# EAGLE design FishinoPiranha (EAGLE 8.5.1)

## Sheet 1 of 6: SUPPLY
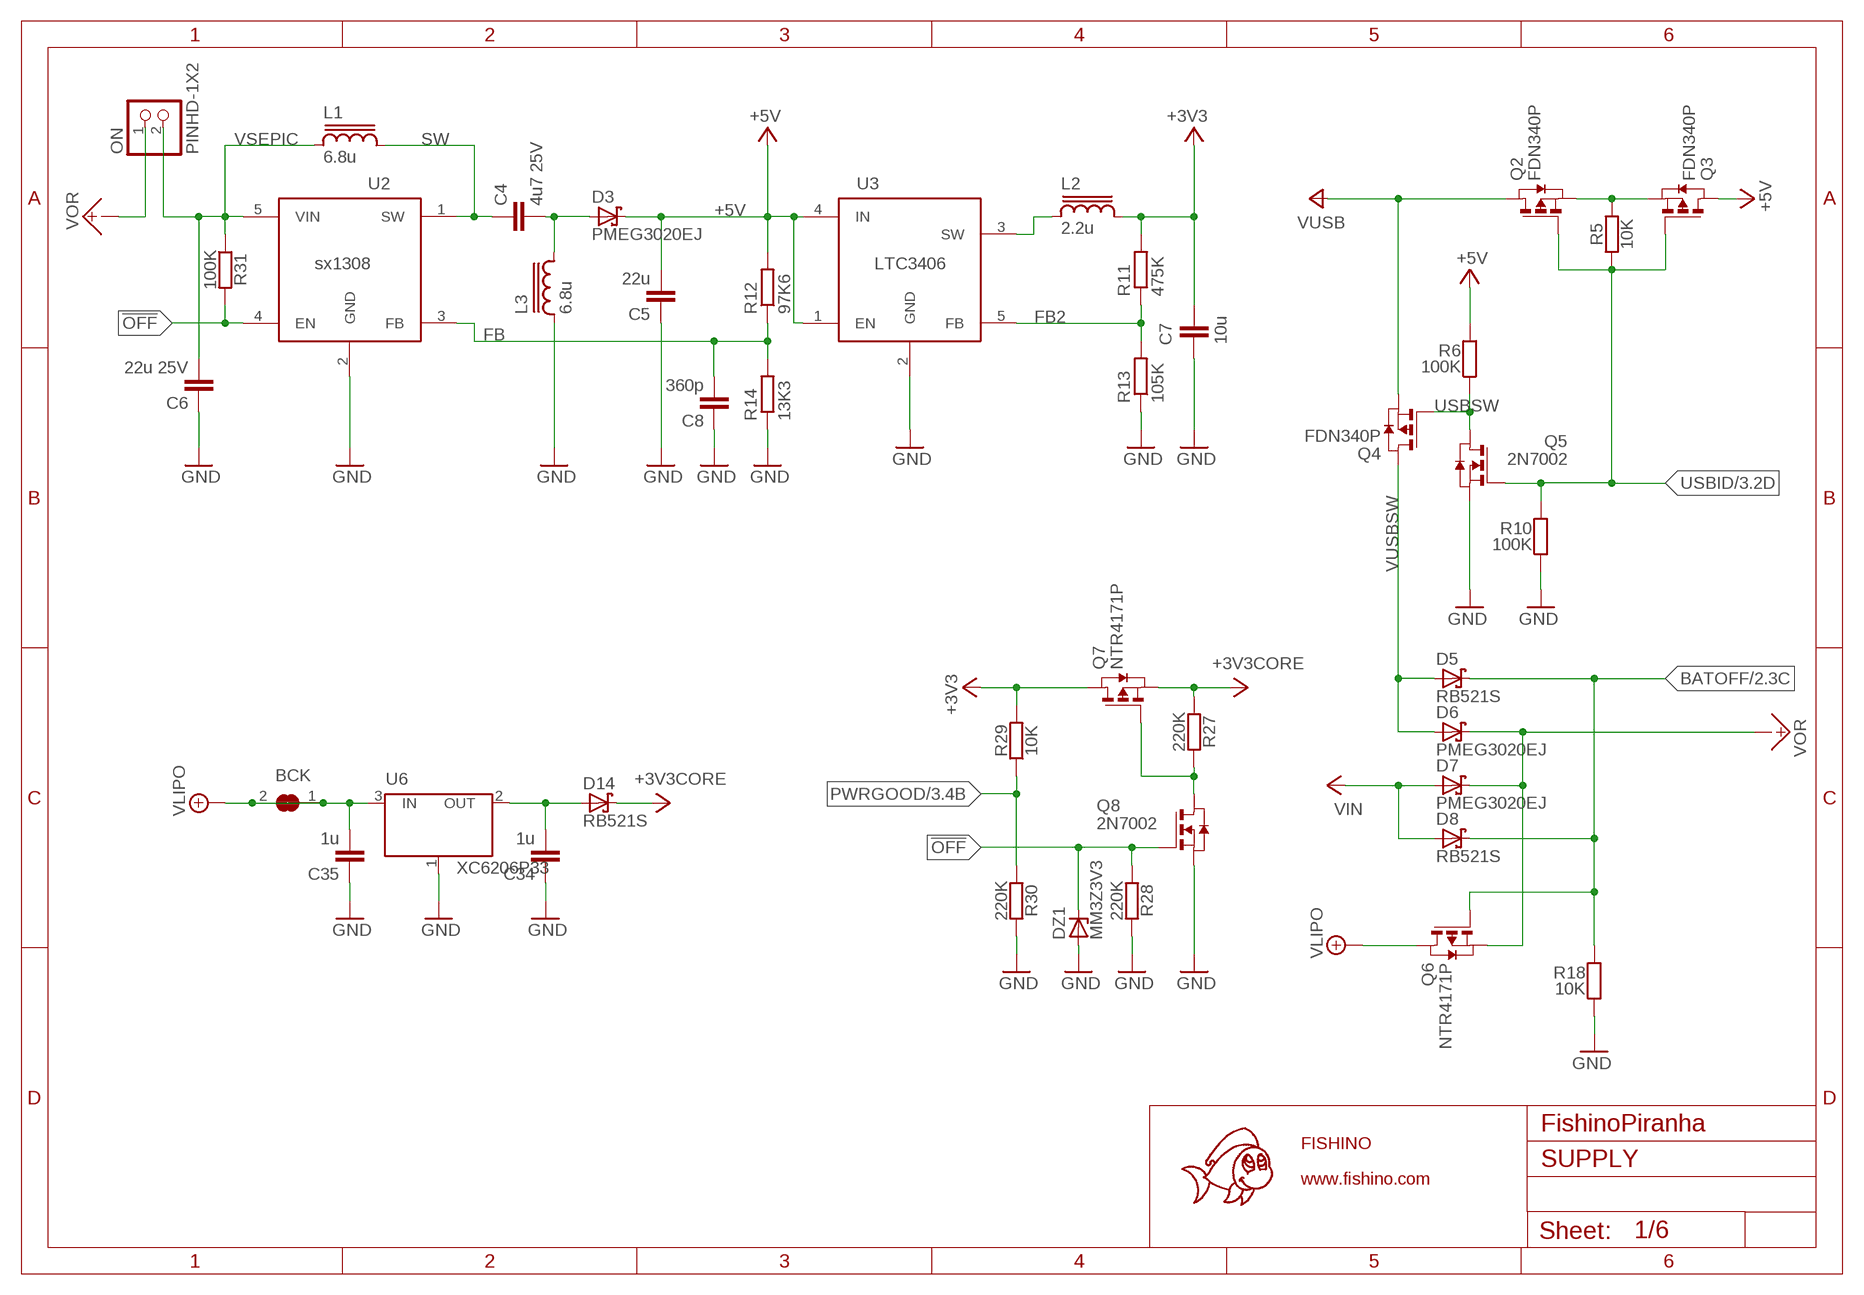
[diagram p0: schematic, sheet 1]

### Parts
BCK  SJ  [SJ]
C4  4u7 25V  C0603-ROUND  [C0603-ROUND]
C5  22u  C0603-ROUND  [C0603-ROUND]
C6  22u 25V  C0603-ROUND  [C0603-ROUND]
C7  10u  C0603-ROUND  [C0603-ROUND]
C8  360p  C0603-ROUND  [C0603-ROUND]
C34  1u  C0603-ROUND  [C0603-ROUND]
C35  1u  C0603-ROUND  [C0603-ROUND]
D3  PMEG3020EJ  [SOD-323]
D5  RB521S  [SOD523]
D6  PMEG3020EJ  [SOD-323]
D7  PMEG3020EJ  [SOD-323]
D8  RB521S  [SOD523]
D14  RB521S  [SOD523]
DZ1  MM3Z3V3  [SOD-323]
L1  6.8u  LSWPA4030S  [SWPA4030S]
L2  2.2u  LCD32  [CD32]
L3  6.8u  LSWPA4030S  [SWPA4030S]
ON  PINHD-1X2  [1X02M]
Q2  FDN340P  PMOSSOT23  [SOT23]
Q3  FDN340P  PMOSSOT23  [SOT23]
Q4  FDN340P  PMOSSOT23  [SOT23]
Q5  2N7002  [SOT23]
Q6  NTR4171P  [SOT23]
Q7  NTR4171P  [SOT23]
Q8  2N7002  [SOT23]
R5  10K  R0603-ROUND  [R0603-ROUND]
R6  100K  R0603-ROUND  [R0603-ROUND]
R10  100K  R0603-ROUND  [R0603-ROUND]
R11  475K  R0603-ROUND  [R0603-ROUND]
R12  97K6  R0603-ROUND  [R0603-ROUND]
R13  105K  R0603-ROUND  [R0603-ROUND]
R14  13K3  R0603-ROUND  [R0603-ROUND]
R18  10K  R0603-ROUND  [R0603-ROUND]
R27  220K  R0603-ROUND  [R0603-ROUND]
R28  220K  R0603-ROUND  [R0603-ROUND]
R29  10K  R0603-ROUND  [R0603-ROUND]
R30  220K  R0603-ROUND  [R0603-ROUND]
R31  100K  R0603-ROUND  [R0603-ROUND]
U2  SX1308  [SOT23-6L]
U3  LC3406  [SOT23-5]
U6  XC6206P33  [SOT23-3]

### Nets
!OFF: DZ1.C Q8.1(G) R28.1 R31.2 U2.4(EN) ; also sheet 3
+3V3: C7.2 L2.2 Q7.3(D) R11.2 R29.2 ; also sheet 3,4,5,6
+3V3CORE: D14.C Q7.2(S) R27.1 ; also sheet 3,5,6
+5V: C5.2 D3.C Q3.3(D) R6.2 R12.2 U3.1(EN) U3.4(IN) ; also sheet 2,6
BATOFF: D5.C D8.C Q6.1(G) R18.2 ; also sheet 2
FB: C8.2 R12.1 R14.2 U2.3(FB)
FB2: R11.1 R13.2 U3.5(FB)
GND [gnd]: C5.1 C6.1 C7.1 C8.1 C34.1 C35.1 DZ1.A L3.P$1 Q5.2(S) Q8.2(S) R10.1 R13.1 R14.1 R18.1 R28.2 R30.2 U2.2(GND) U3.2(GND) U6.1(GND/ADJ) ; also sheet 2,3,4,5,6
N17690335: Q2.2(S) Q3.2(S) R5.2
N$1: C34.2 D14.A U6.2(OUT)
N$24: C4.2 D3.A L3.P$2
N$34: Q7.1(G) Q8.3(D) R27.2
PWRGOOD: R29.1 R30.1 ; also sheet 3
SW: C4.1 L1.P$2 U2.1(SW)
SW2: L2.1 U3.3(SW)
USBID: Q2.1(G) Q3.1(G) Q5.1(G) R5.1 R10.2 ; also sheet 3,6
USBSW: Q4.1(G) Q5.3(D) R6.1
VIN: D7.A D8.A ; also sheet 6
VLIPO: BCK.1 BCK.2 C35.2 Q6.3(D) U6.3(IN) ; also sheet 2
VOR [power]: D6.C D7.C ON.1 Q6.2(S)
VSEPIC [power]: C6.2 L1.P$1 ON.2 R31.1 U2.5(VIN)
VUSB: Q2.3(D) Q4.2(S) ; also sheet 3,6
VUSBSW: D5.A D6.A Q4.3(D)

## Sheet 2 of 6: BATTERY CHARGER
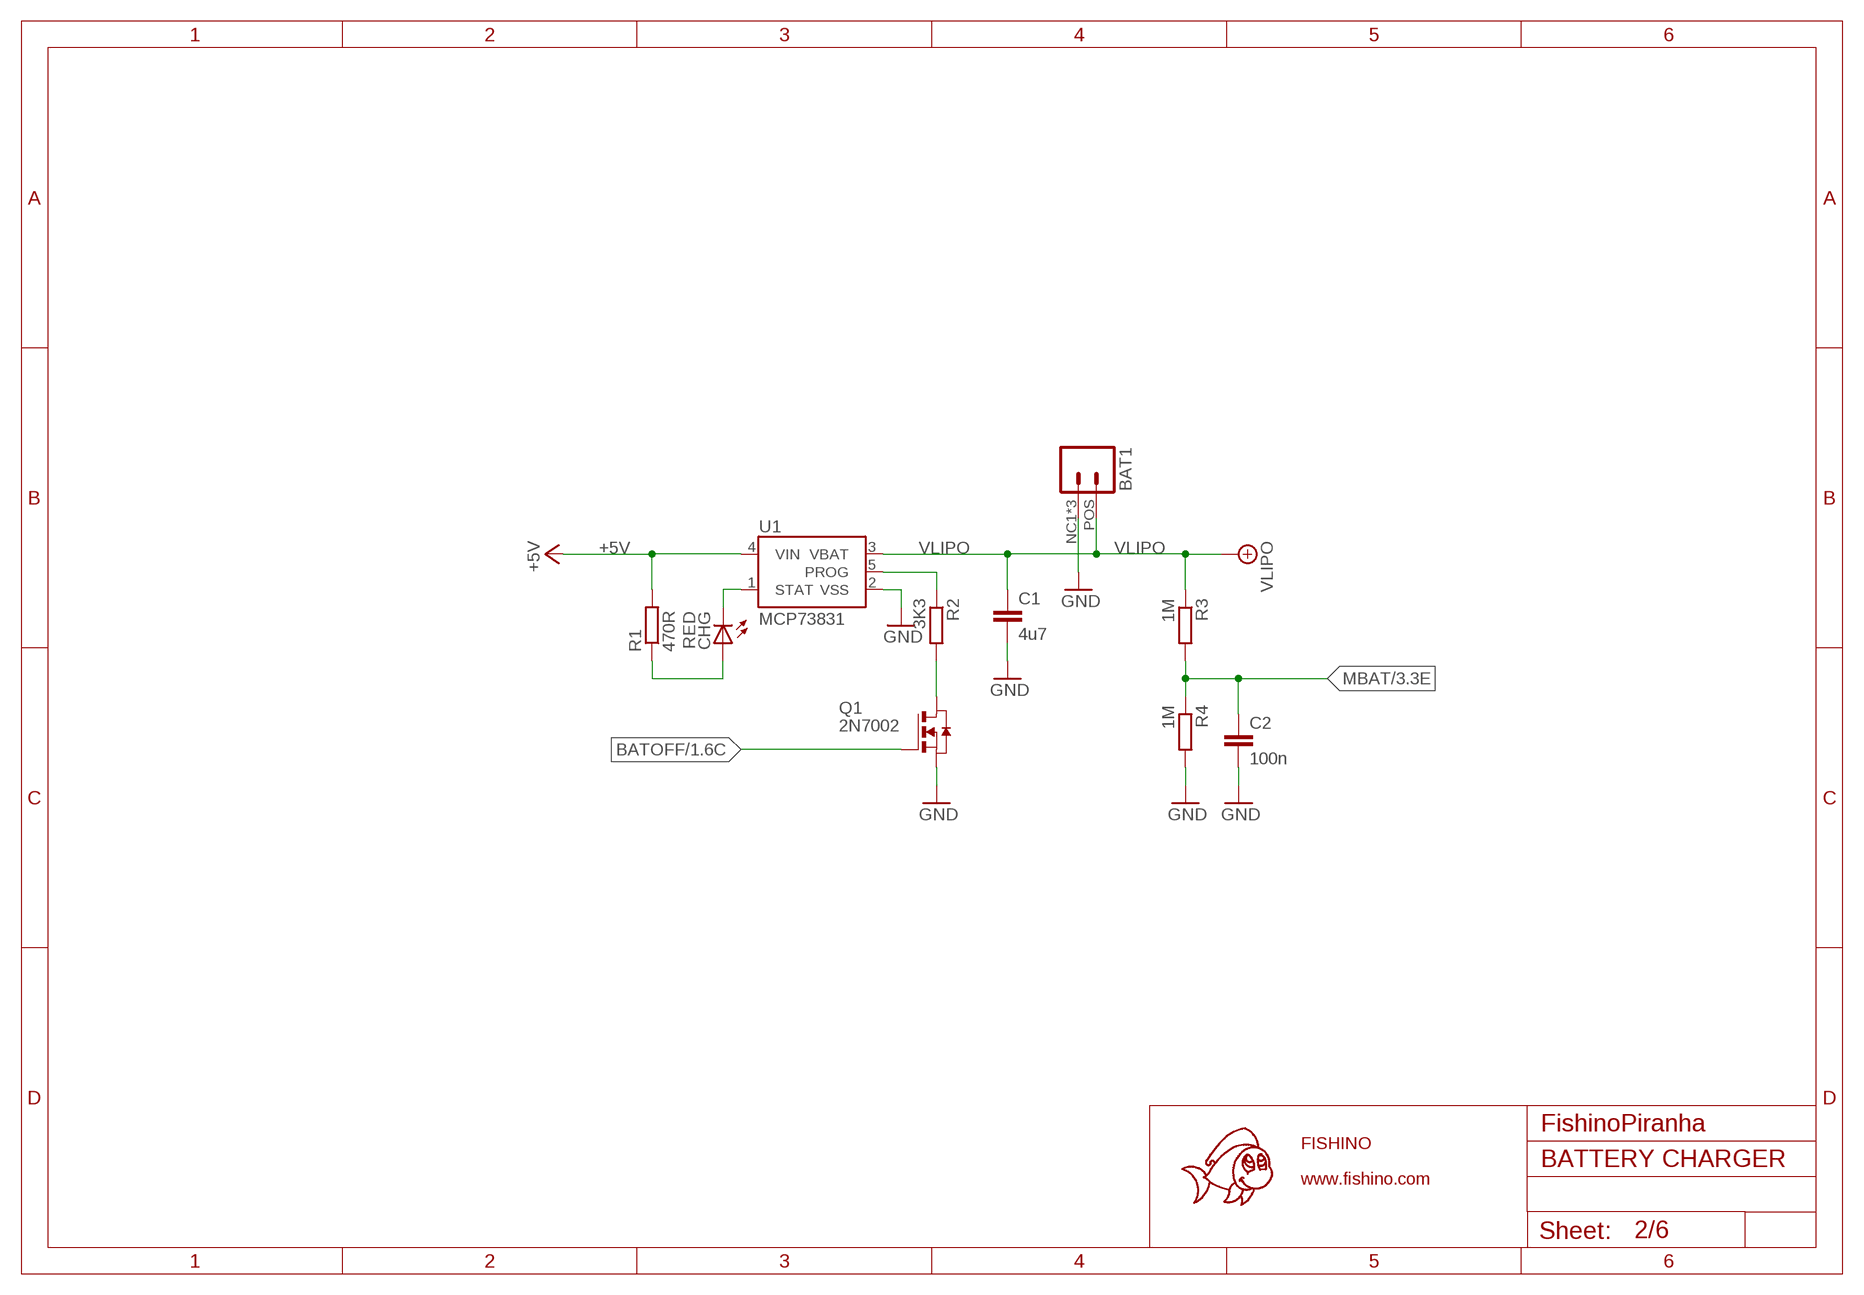
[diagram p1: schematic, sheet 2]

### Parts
BAT1  MO2-JST-2-2MM-SMT-STANDARD  [JST-2-SMD-STANDARD]
C1  4u7  C0603-ROUND  [C0603-ROUND]
C2  100n  C0603-ROUND  [C0603-ROUND]
CHG  RED  LED0603  [CHIPLED_0603]
Q1  2N7002  [SOT23]
R1  470R  R0603-ROUND  [R0603-ROUND]
R2  3K3  R0603-ROUND  [R0603-ROUND]
R3  1M  R0603-ROUND  [R0603-ROUND]
R4  1M  R0603-ROUND  [R0603-ROUND]
U1  MCP73831  [SOT23-5]

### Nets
+5V: R1.2 U1.4(VIN) ; also sheet 1,6
BATOFF: Q1.1(G) ; also sheet 1
GND [gnd]: BAT1.NC1(NEG) BAT1.NC2(NEG) BAT1.NEG C1.2 C2.2 Q1.2(S) R4.2 U1.2(VSS) ; also sheet 1,3,4,5,6
MBAT: C2.1 R3.2 R4.1 ; also sheet 3
N$7: Q1.3(D) R2.2
N$20: CHG.A R1.1
PROG: R2.1 U1.5(PROG)
STAT2: CHG.C U1.1(STAT)
VLIPO: BAT1.POS C1.1 R3.1 U1.3(VBAT) ; also sheet 1

## Sheet 3 of 6: CONTROLLER
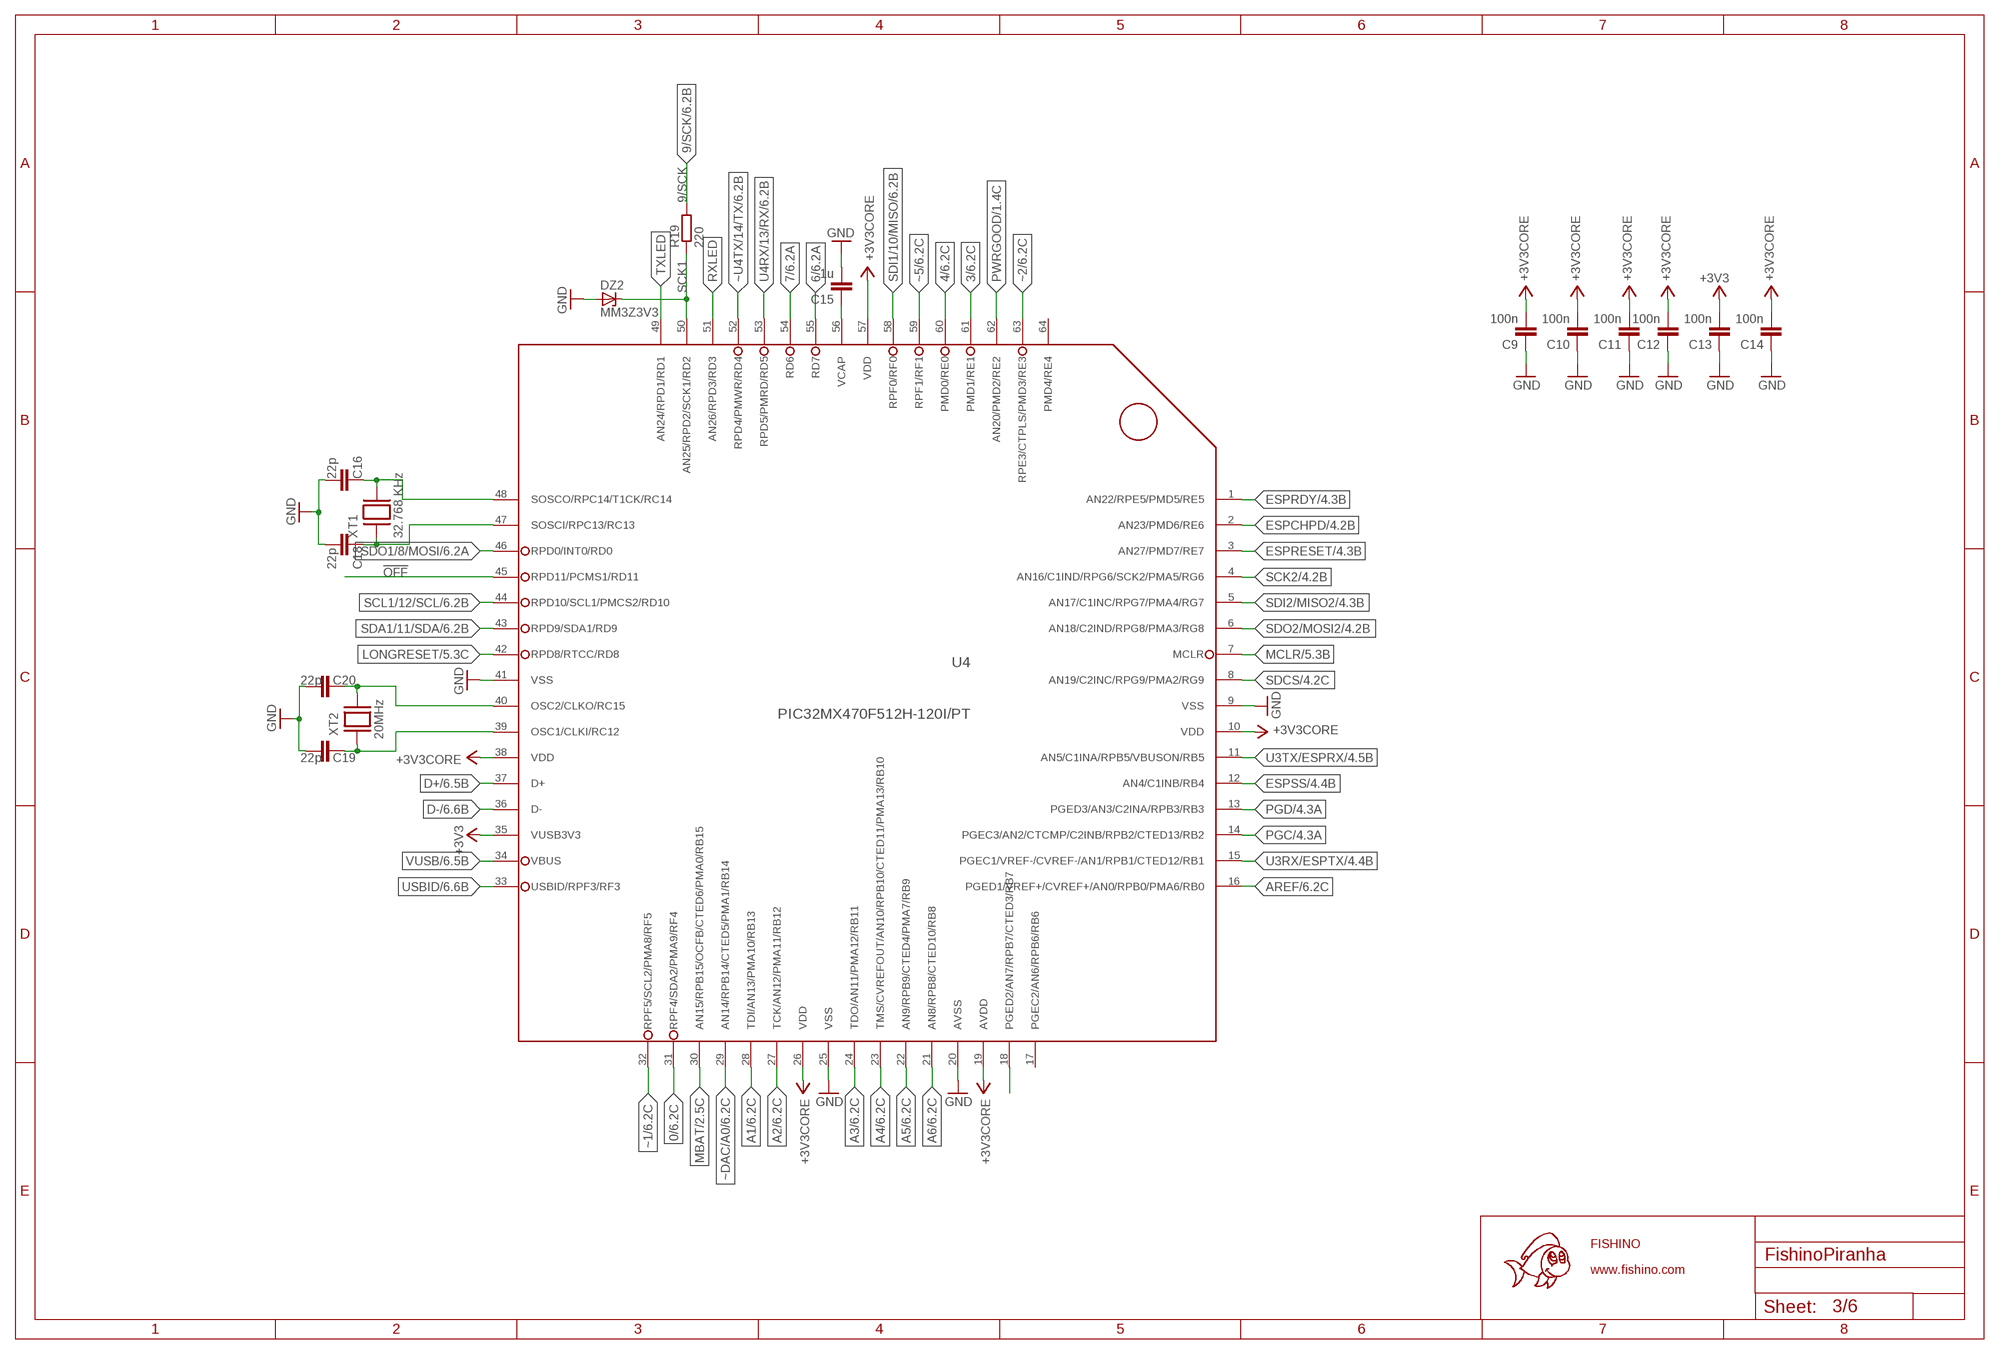
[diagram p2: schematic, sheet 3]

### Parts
C9  100n  C0603-ROUND  [C0603-ROUND]
C10  100n  C0603-ROUND  [C0603-ROUND]
C11  100n  C0603-ROUND  [C0603-ROUND]
C12  100n  C0603-ROUND  [C0603-ROUND]
C13  100n  C0603-ROUND  [C0603-ROUND]
C14  100n  C0603-ROUND  [C0603-ROUND]
C15  1u  C0603-ROUND  [C0603-ROUND]
C16  22p  C0603-ROUND  [C0603-ROUND]
C18  22p  C0603-ROUND  [C0603-ROUND]
C19  22p  C0603-ROUND  [C0603-ROUND]
C20  22p  C0603-ROUND  [C0603-ROUND]
DZ2  MM3Z3V3  [SOD-323]
R19  220  R0603-ROUND  [R0603-ROUND]
U4  PIC32MX470F512H-120I/PT  [TQFP64-10X10]
XT1  32.768 KHz  XTAL/SFC145  [FC145]
XT2  20MHz  XTAL/SIQG2520  [IQG2520]

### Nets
0: U4.31(RPF4/SDA2/PMA9/RF4) ; also sheet 6
3: U4.61(PMD1/RE1) ; also sheet 6
4: U4.60(PMD0/RE0) ; also sheet 6
6: U4.55(RD7) ; also sheet 6
7: U4.54(RD6) ; also sheet 6
9/SCK: R19.2 ; also sheet 6
!OFF: U4.45(RPD11/PCMS1/RD11) ; also sheet 1
+3V3: C13.2 U4.35(VUSB3V3) ; also sheet 1,4,5,6
+3V3CORE: C9.2 C10.2 C11.2 C12.2 C14.2 U4.10(VDD) U4.19(AVDD) U4.26(VDD) U4.38(VDD) U4.57(VDD) ; also sheet 1,5,6
A1: U4.28(TDI/AN13/PMA10/RB13) ; also sheet 6
A2: U4.27(TCK/AN12/PMA11/RB12) ; also sheet 6
A3: U4.24(TDO/AN11/PMA12/RB11) ; also sheet 6
A4: U4.23(TMS/CVREFOUT/AN10/RPB10/CTED11/PMA13/RB10) ; also sheet 6
A5: U4.22(AN9/RPB9/CTED4/PMA7/RB9) ; also sheet 6
A6: U4.21(AN8/RPB8/CTED10/RB8) ; also sheet 6
AREF: U4.16(PGED1/VREF+/CVREF+/AN0/RPB0/PMA6/RB0) ; also sheet 6
D+: U4.37(D+) ; also sheet 6
D-: U4.36(D-) ; also sheet 6
ESPBMODE: U4.18(PGED2/AN7/RPB7/CTED3/RB7) ; also sheet 4
ESPCHPD: U4.2(AN23/PMD6/RE6) ; also sheet 4
ESPRDY: U4.1(AN22/RPE5/PMD5/RE5) ; also sheet 4
ESPRESET: U4.3(AN27/PMD7/RE7) ; also sheet 4
ESPSS: U4.12(AN4/C1INB/RB4) ; also sheet 4
GND [gnd]: C9.1 C10.1 C11.1 C12.1 C13.1 C14.1 C15.2 C16.2 C18.2 C19.2 C20.2 DZ2.A U4.9(VSS) U4.20(AVSS) U4.25(VSS) U4.41(VSS) ; also sheet 1,2,4,5,6
LONGRESET: U4.42(RPD8/RTCC/RD8) ; also sheet 5
MBAT: U4.30(AN15/RPB15/OCFB/CTED6/PMA0/RB15) ; also sheet 2
MCLR: U4.7(MCLR) ; also sheet 5,6
N$2: C15.1 U4.56(VCAP)
N$5: C18.1 U4.47(SOSCI/RPC13/RC13) XT1.P$1
N$6: C16.1 U4.48(SOSCO/RPC14/T1CK/RC14) XT1.P$2
OSC1: C19.1 U4.39(OSC1/CLKI/RC12) XT2.P$3
OSC2: C20.1 U4.40(OSC2/CLKO/RC15) XT2.P$1
PGC: U4.14(PGEC3/AN2/CTCMP/C2INB/RPB2/CTED13/RB2) ; also sheet 4,6
PGD: U4.13(PGED3/AN3/C2INA/RPB3/RB3) ; also sheet 4,6
PWRGOOD: U4.62(AN20/PMD2/RE2) ; also sheet 1
RXLED: U4.51(AN26/RPD3/RD3) ; also sheet 5
SCK1: DZ2.C R19.1 U4.50(AN25/RPD2/SCK1/RD2)
SCK2: U4.4(AN16/C1IND/RPG6/SCK2/PMA5/RG6) ; also sheet 4
SCL1/12/SCL: U4.44(RPD10/SCL1/PMCS2/RD10) ; also sheet 6
SDA1/11/SDA: U4.43(RPD9/SDA1/RD9) ; also sheet 6
SDCS: U4.8(AN19/C2INC/RPG9/PMA2/RG9) ; also sheet 4
SDI1/10/MISO: U4.58(RPF0/RF0) ; also sheet 6
SDI2/MISO2: U4.5(AN17/C1INC/RPG7/PMA4/RG7) ; also sheet 4
SDO1/8/MOSI: U4.46(RPD0/INT0/RD0) ; also sheet 6
SDO2/MOSI2: U4.6(AN18/C2IND/RPG8/PMA3/RG8) ; also sheet 4
TXLED: U4.49(AN24/RPD1/RD1) ; also sheet 5
U3RX/ESPTX: U4.15(PGEC1/VREF-/CVREF-/AN1/RPB1/CTED12/RB1) ; also sheet 4
U3TX/ESPRX: U4.11(AN5/C1INA/RPB5/VBUSON/RB5) ; also sheet 4
U4RX/13/RX: U4.53(RPD5/PMRD/RD5) ; also sheet 6
USBID: U4.33(USBID/RPF3/RF3) ; also sheet 1,6
VUSB: U4.34(VBUS) ; also sheet 1,6
~1: U4.32(RPF5/SCL2/PMA8/RF5) ; also sheet 6
~2: U4.63(RPE3/CTPLS/PMD3/RE3) ; also sheet 6
~5: U4.59(RPF1/RF1) ; also sheet 6
~DAC/A0: U4.29(AN14/RPB14/CTED5/PMA1/RB14) ; also sheet 6
~U4TX/14/TX: U4.52(RPD4/PMWR/RD4) ; also sheet 6
Unconnected: U4.17(PGEC2/AN6/RPB6/RB6) U4.64(PMD4/RE4)

## Sheet 4 of 6: WIFI AND SD
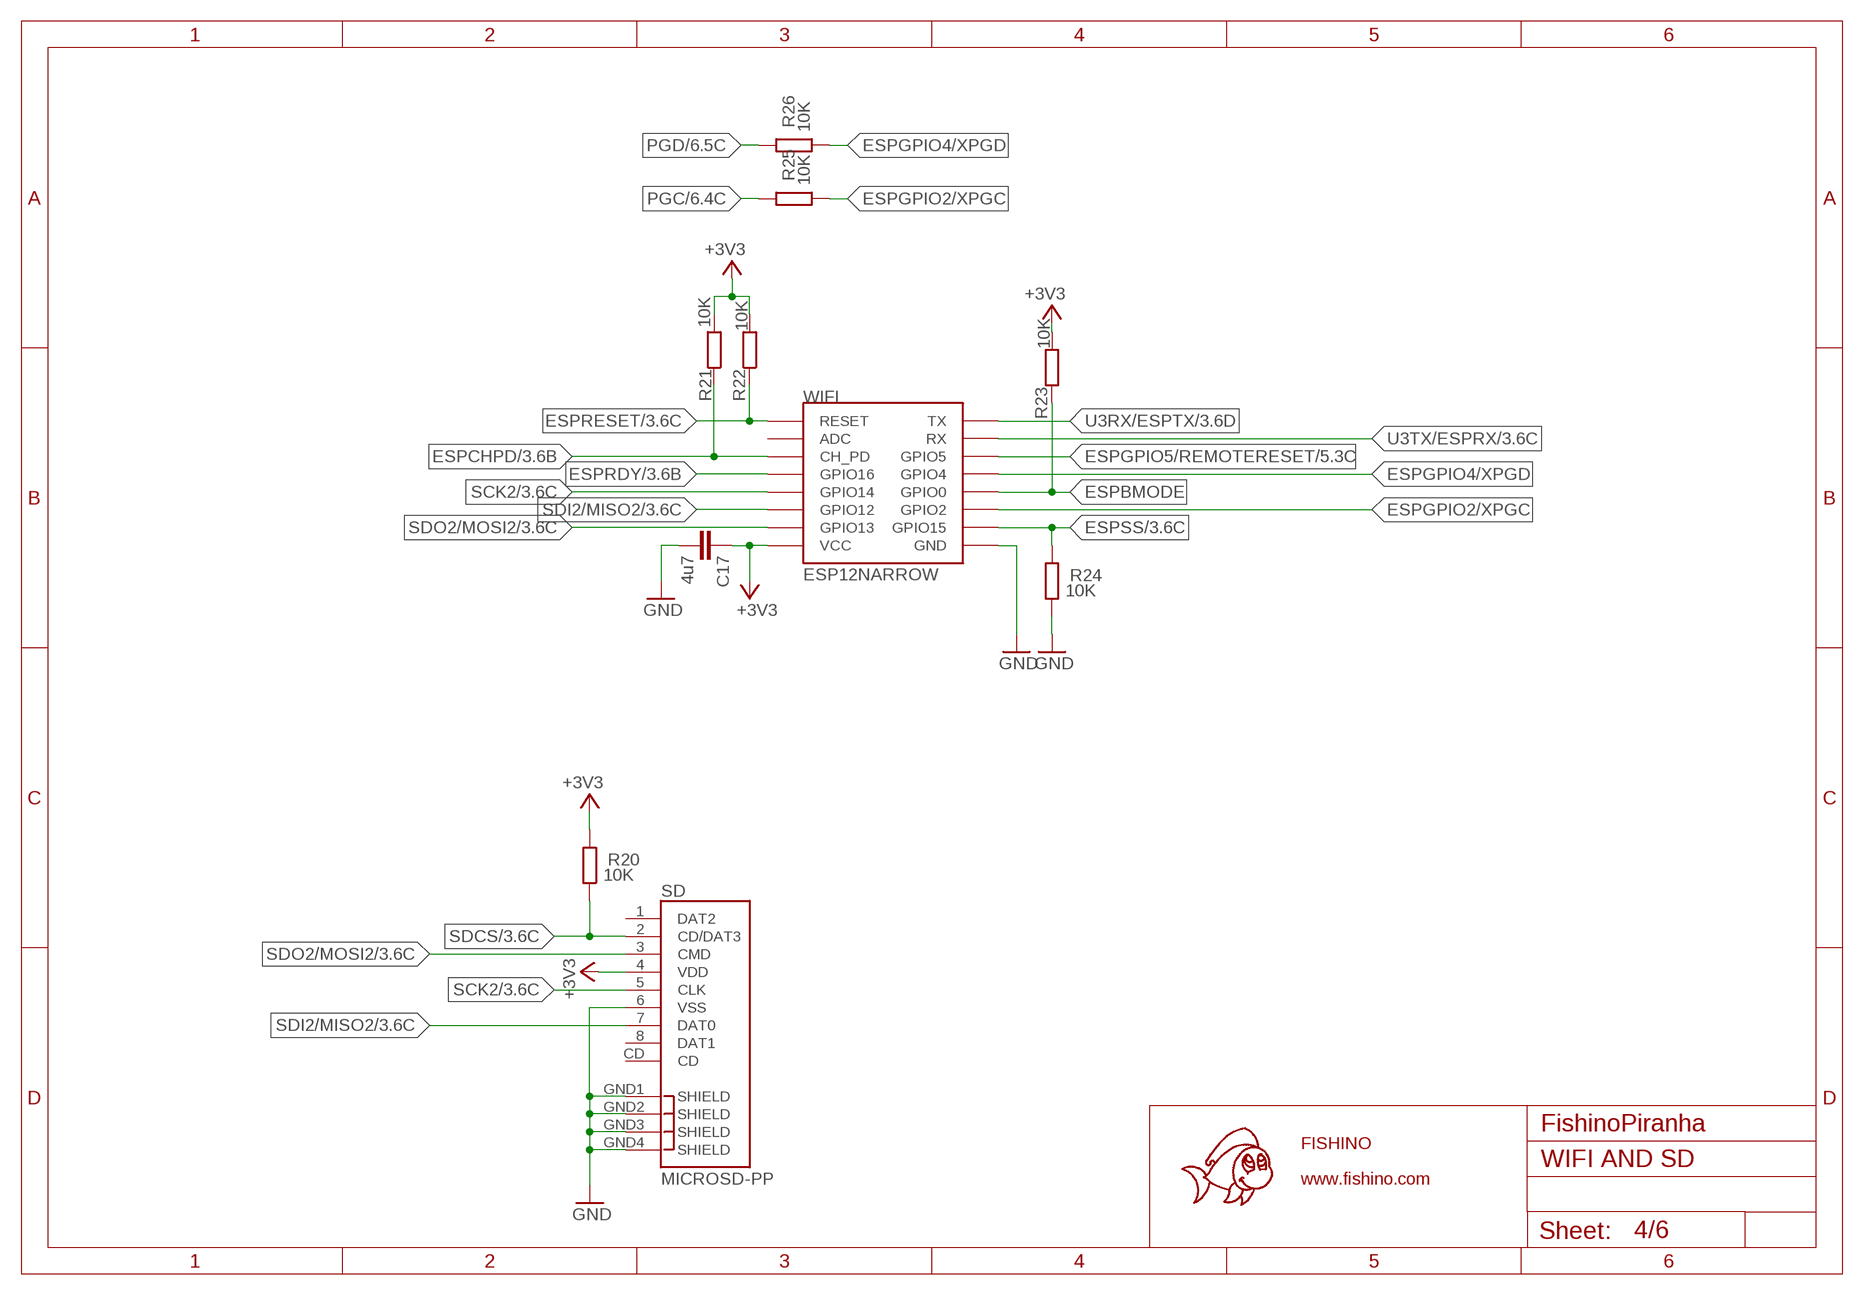
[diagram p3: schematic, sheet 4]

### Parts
C17  4u7  C0603-ROUND  [C0603-ROUND]
R20  10K  R0603-ROUND  [R0603-ROUND]
R21  10K  R0603-ROUND  [R0603-ROUND]
R22  10K  R0603-ROUND  [R0603-ROUND]
R23  10K  R0603-ROUND  [R0603-ROUND]
R24  10K  R0603-ROUND  [R0603-ROUND]
R25  10K  R0603-ROUND  [R0603-ROUND]
R26  10K  R0603-ROUND  [R0603-ROUND]
SD  MICROSD-PP  [MICROSD-PUSHPULL]
WIFI  ESP12NARROW  [ESP12SMD-NARROW]

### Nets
+3V3: C17.1 R20.2 R21.2 R22.2 R23.2 SD.4(VDD) WIFI.VCC ; also sheet 1,3,5,6
ESPBMODE: R23.1 WIFI.GPIO0 ; also sheet 3
ESPCHPD: R21.1 WIFI.CH_PD ; also sheet 3
ESPGPIO2/XPGC: R25.1 WIFI.GPIO2
ESPGPIO4/XPGD: R26.1 WIFI.GPIO4
ESPGPIO5/REMOTERESET: WIFI.GPIO5 ; also sheet 5
ESPRDY: WIFI.GPIO16 ; also sheet 3
ESPRESET: R22.1 WIFI.RESET ; also sheet 3
ESPSS: R24.2 WIFI.GPIO15 ; also sheet 3
GND [gnd]: C17.2 R24.1 SD.6(VSS) SD.GND1(SHIELD) SD.GND2(SHIELD) SD.GND3(SHIELD) SD.GND4(SHIELD) WIFI.GND ; also sheet 1,2,3,5,6
PGC: R25.2 ; also sheet 3,6
PGD: R26.2 ; also sheet 3,6
SCK2: SD.5(CLK) WIFI.GPIO14 ; also sheet 3
SDCS: R20.1 SD.2(CD/DAT3) ; also sheet 3
SDI2/MISO2: SD.7(DAT0) WIFI.GPIO12 ; also sheet 3
SDO2/MOSI2: SD.3(CMD) WIFI.GPIO13 ; also sheet 3
U3RX/ESPTX: WIFI.TX ; also sheet 3
U3TX/ESPRX: WIFI.RX ; also sheet 3
Unconnected: SD.1(DAT2) SD.8(DAT1) SD.CD WIFI.ADC

## Sheet 5 of 6: RESET AND LEDS
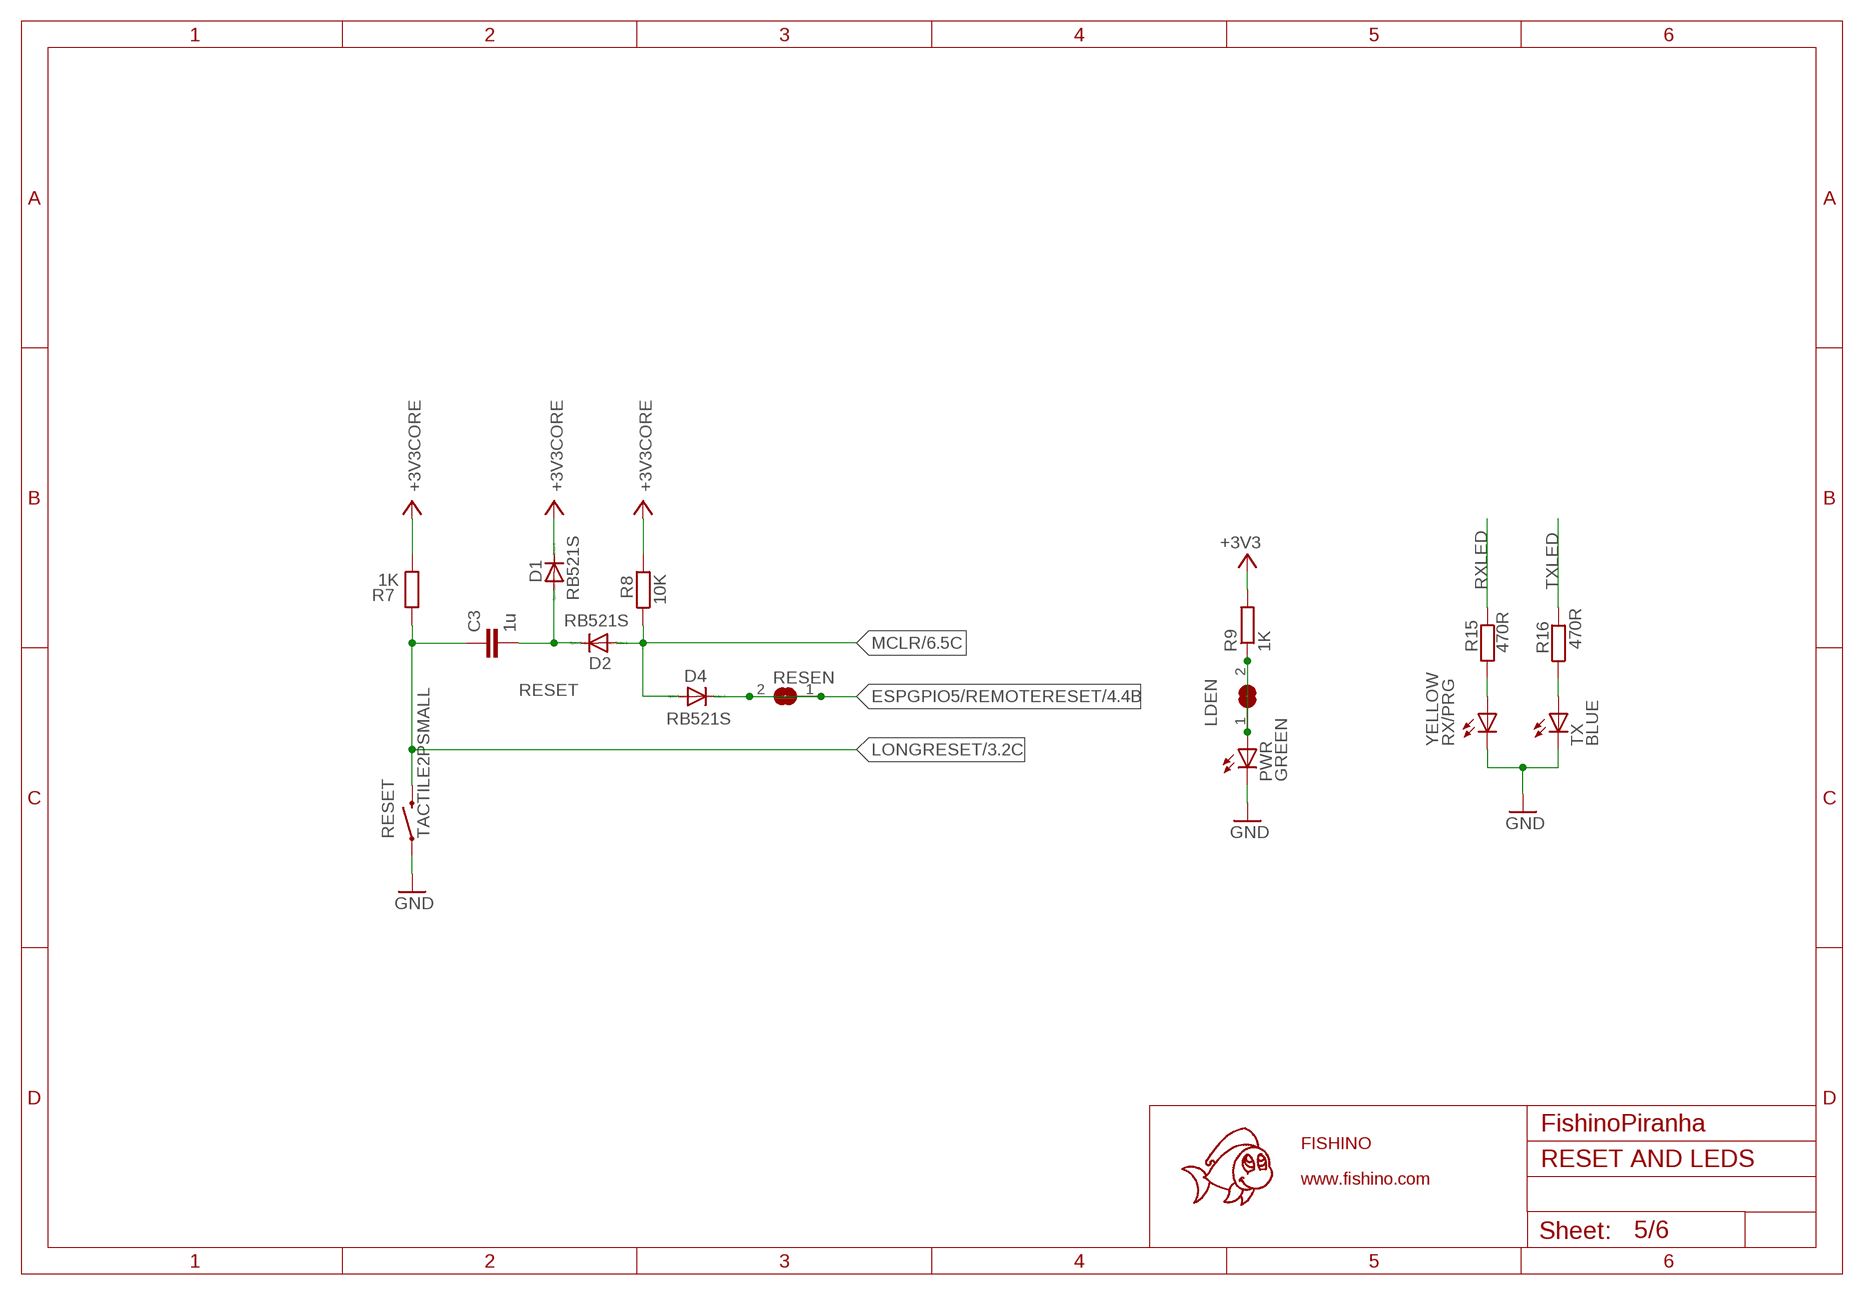
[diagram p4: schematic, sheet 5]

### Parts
C3  1u  C0603-ROUND  [C0603-ROUND]
D1  RB521S  DIODE-SOD523  [SOD523]
D2  RB521S  DIODE-SOD523  [SOD523]
D4  RB521S  DIODE-SOD523  [SOD523]
LDEN  SJ  [SJ]
PWR  GREEN  LED0603  [CHIPLED_0603]
R7  1K  R0603-ROUND  [R0603-ROUND]
R8  10K  R0603-ROUND  [R0603-ROUND]
R9  1K  R0603-ROUND  [R0603-ROUND]
R15  470R  R0603-ROUND  [R0603-ROUND]
R16  470R  R0603-ROUND  [R0603-ROUND]
RESEN  SJ  [SJ]
RESET  TACTILE2PSMALL  [TACTILE-SWITCH-1101NE]
RX/PRG  YELLOW  LED0603  [CHIPLED_0603]
TX  BLUE  LED0603  [CHIPLED_0603]

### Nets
+3V3: R9.2 ; also sheet 1,3,4,6
+3V3CORE: D1.C R7.1 R8.2 ; also sheet 1,3,6
ESPGPIO5/REMOTERESET: D4.C RESEN.1 RESEN.2 ; also sheet 4
GND [gnd]: PWR.C RESET.1 RX/PRG.C TX.C ; also sheet 1,2,3,4,6
LONGRESET: C3.1 R7.2 RESET.2 ; also sheet 3
MCLR: D2.A D4.A R8.1 ; also sheet 3,6
N$10: R16.1 TX.A
N$13: LDEN.1 LDEN.2 PWR.A R9.1
N$14: R15.2 RX/PRG.A
RESET: C3.2 D1.A D2.C ; also sheet 6
RXLED: R15.1 ; also sheet 3
TXLED: R16.2 ; also sheet 3

## Sheet 6 of 6: HEADERS
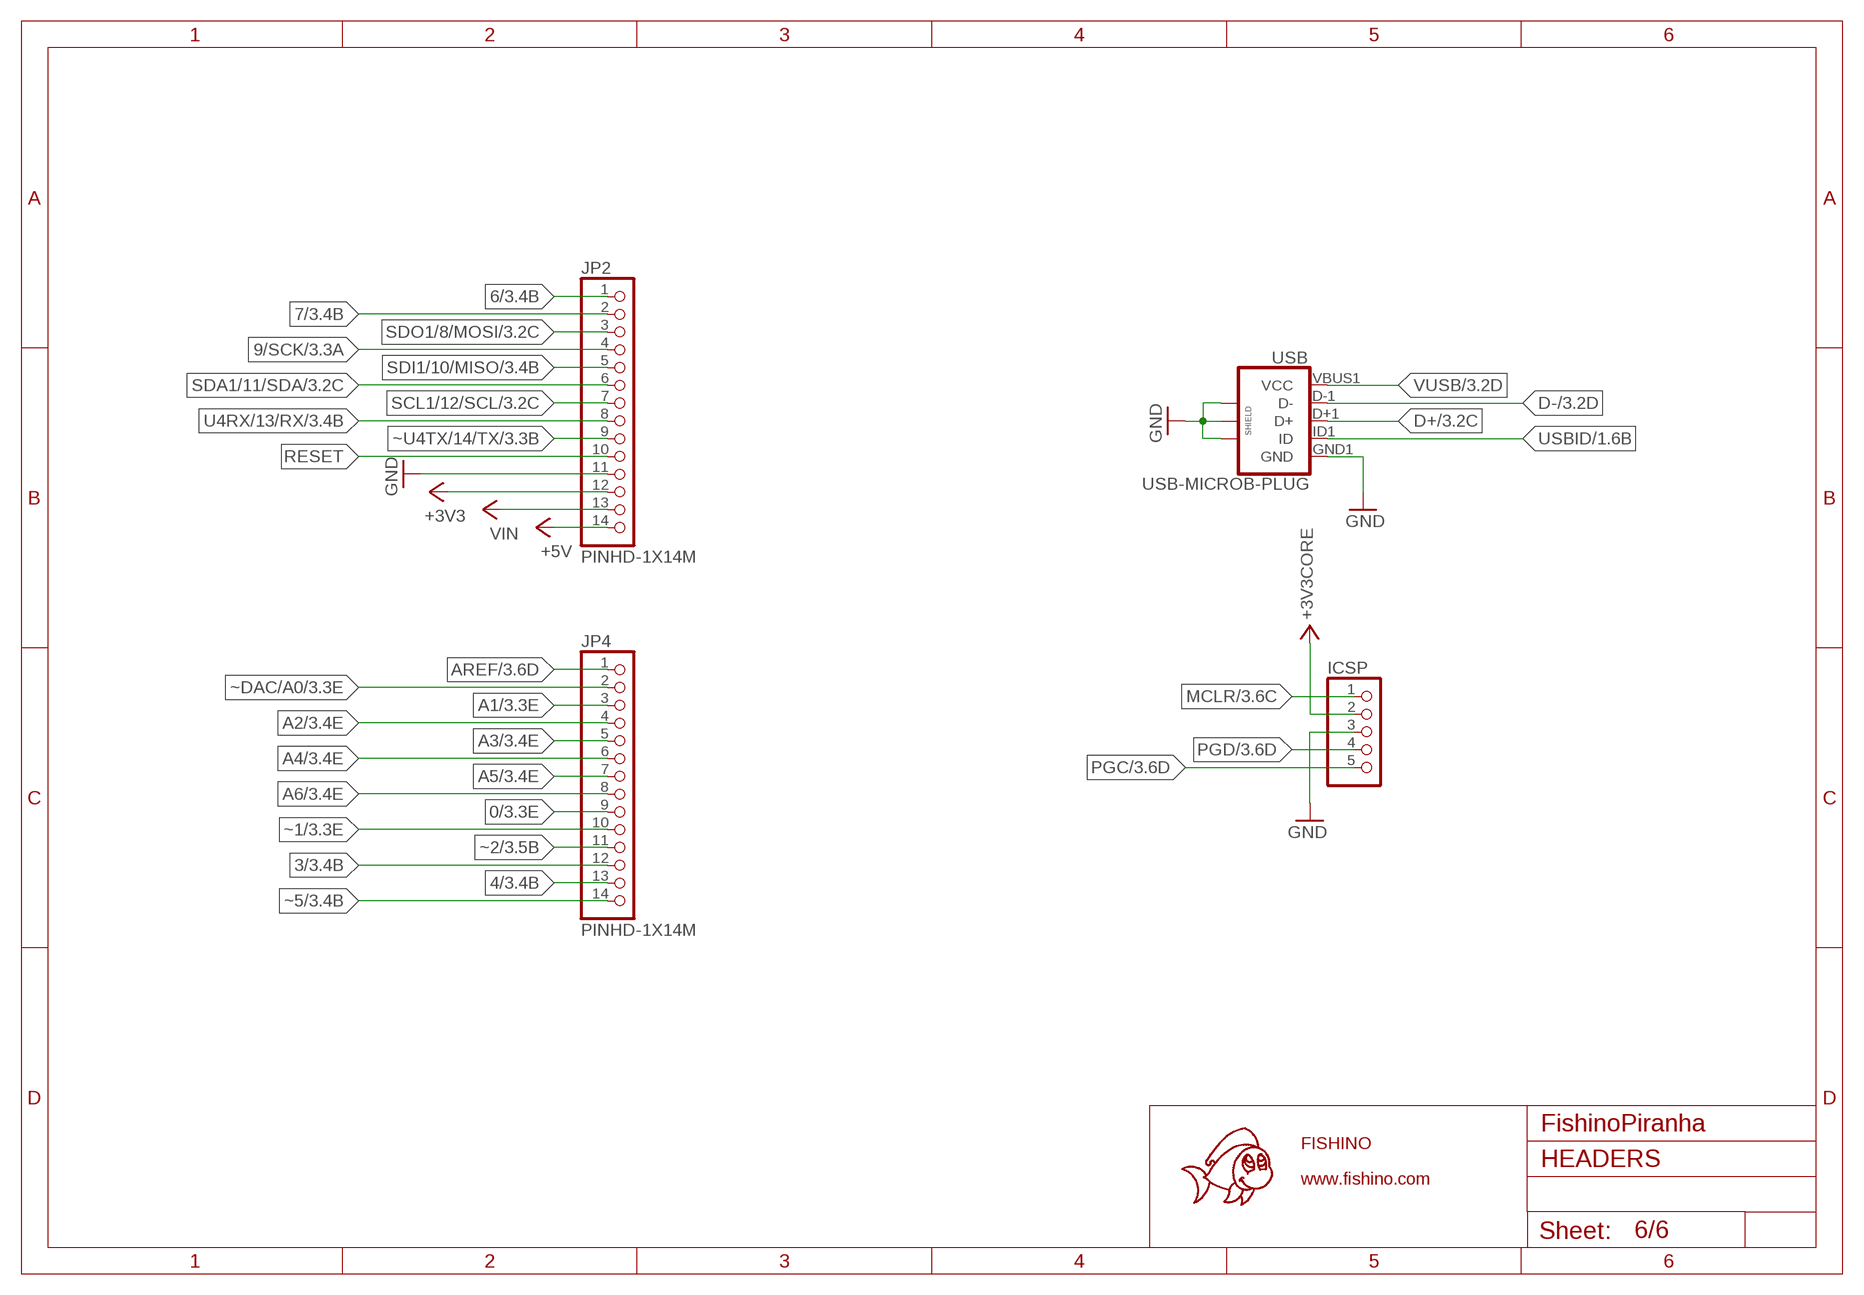
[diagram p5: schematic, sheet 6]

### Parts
ICSP  PINHD-1X5  [1X05M]
JP2  PINHD-1X14M  [1X14M]
JP4  PINHD-1X14M  [1X14M]
USB  USB-MICROB-PLUG  [USB-B-MICRO-SMD_V03]

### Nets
0: JP4.9 ; also sheet 3
3: JP4.12 ; also sheet 3
4: JP4.13 ; also sheet 3
6: JP2.1 ; also sheet 3
7: JP2.2 ; also sheet 3
9/SCK: JP2.4 ; also sheet 3
+3V3: JP2.12 ; also sheet 1,3,4,5
+3V3CORE: ICSP.2 ; also sheet 1,3,5
+5V: JP2.14 ; also sheet 1,2
A1: JP4.3 ; also sheet 3
A2: JP4.4 ; also sheet 3
A3: JP4.5 ; also sheet 3
A4: JP4.6 ; also sheet 3
A5: JP4.7 ; also sheet 3
A6: JP4.8 ; also sheet 3
AREF: JP4.1 ; also sheet 3
D+: USB.D+1(D+) ; also sheet 3
D-: USB.D-1(D-) ; also sheet 3
GND [gnd]: ICSP.3 JP2.11 USB.GND1(GND) USB.SHIELD1 USB.SHIELD2 USB.SHIELD3 ; also sheet 1,2,3,4,5
MCLR: ICSP.1 ; also sheet 3,5
PGC: ICSP.5 ; also sheet 3,4
PGD: ICSP.4 ; also sheet 3,4
RESET: JP2.10 ; also sheet 5
SCL1/12/SCL: JP2.7 ; also sheet 3
SDA1/11/SDA: JP2.6 ; also sheet 3
SDI1/10/MISO: JP2.5 ; also sheet 3
SDO1/8/MOSI: JP2.3 ; also sheet 3
U4RX/13/RX: JP2.8 ; also sheet 3
USBID: USB.ID1(ID) ; also sheet 1,3
VIN: JP2.13 ; also sheet 1
VUSB: USB.VBUS1(VCC) ; also sheet 1,3
~1: JP4.10 ; also sheet 3
~2: JP4.11 ; also sheet 3
~5: JP4.14 ; also sheet 3
~DAC/A0: JP4.2 ; also sheet 3
~U4TX/14/TX: JP2.9 ; also sheet 3

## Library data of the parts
BAT1 = Max-Connectors:MO2-JST-2-2MM-SMT-STANDARD
BCK LDEN RESEN = jumper:SJ: SMD solder JUMPER
C1-C20 C34 C35 = Max-RCL:C
CHG PWR RX/PRG TX = Max-Led:LED
D1 D2 D4 = diode:DIODE-: DIODE
D3 D6 D7 = Max-Diodes:PMEG3020
D5 D8 D14 = Max-Diodes:RB521S
DZ1 DZ2 = Max-Diodes:MM3Z3V3
ICSP = Max-PinHead:PINHD-1X5: 5 Pin header
JP2 JP4 = Max-PinHead:PINHD-1X14
L1-L3 = Max-RCL:L
ON = Max-PinHead:PINHD-1X2
Q1 Q5 Q8 = Max-Mosfets:2N7002
Q2-Q4 = Max-Mosfets:PMOSSOT23: MOS FET
Q6 Q7 = Max-Mosfets:NTR4171P
R1-R16 R18-R31 = Max-RCL:R
RESET = Max-Switches:TACTILE2P
SD = Max-Connectors:MICROSD-PP
U1 = Max-LinearRegulators:MCP73831: Microchip's MCP73831 Miniature single cell, fully integrated Li-Ion, Li-polymer charge management controller http://ww1.microchip.com/downloads/en/DeviceDoc/21984a.pdf
U2 = Max-SwitchingRegulators:SX1308
U3 = Max-SwitchingRegulators:LC3406
U4 = Max-PIC:PIC32MX470F512H-120
U6 = Max-LinearRegulators:XC6206P
USB = Max-Connectors:USB-MICROB-PLUG
WIFI = Max-ESPModules:ESP12: ESP8266 Wifi module 12
XT1 XT2 = Max-Crystals:XTAL/S: CRYSTAL

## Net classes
0 default: width 0.152 mm, clearance 0.152 mm
1 power: width 0.254 mm, drill 0.61 mm, clearance 0.203 mm
2 gnd: width 0.254 mm, drill 0.61 mm, clearance 0.203 mm
3 usbvcc: width 0.254 mm, drill 0.61 mm, clearance 0.203 mm

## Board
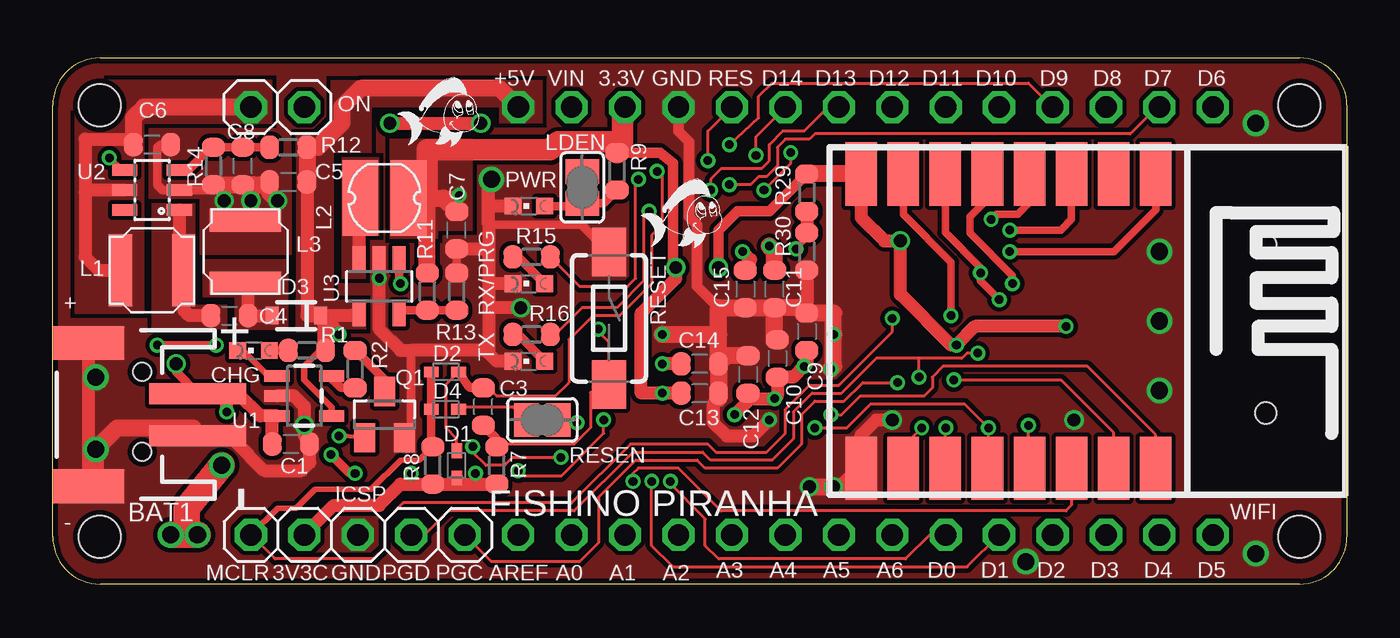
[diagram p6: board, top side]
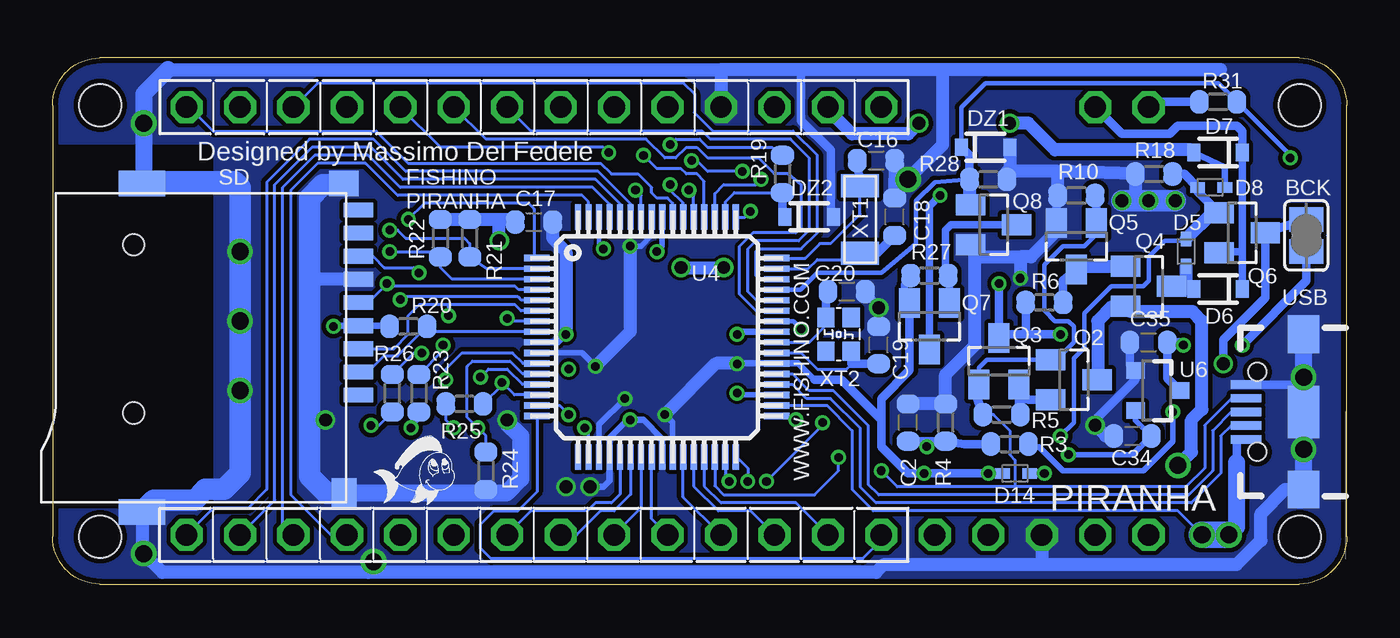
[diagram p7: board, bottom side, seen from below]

Size 61.5 x 25 mm. Coordinates in mm from the lower left corner, seen from the top.
Outline: 59.25,0 2.25,0 arc-90 0,2.25 0,22.75 arc-90 2.25,25 59.25,25 arc-90 61.5,22.75 61.5,2.25 arc-90 59.25,0
Copper layers (1*16): Top 0.035mm / dielectric 1.5mm / Bottom 0.035mm
Design rules "Elecrow_2-layer_eagle_rule": minimum track width 6mil, minimum drill 12mil, track to track 6mil, track to pad 6mil, pad to pad 6mil, via to via 6mil, smd to smd 0mil, copper to edge 10mil, drill to drill 10mil, minimum pad ring 10mil, minimum via ring 6mil, stop-mask expansion 2mil, vias tented up to drill 100mil, thermal gap 10mil
Holes 2 mm at 2.24,2.25 2.24,22.75 59.24,22.75 59.24,2.25
tRestrict: area 54,4.1 to 61.5,20.8
bRestrict: area 53.9,3.6 to 61.5,20.9

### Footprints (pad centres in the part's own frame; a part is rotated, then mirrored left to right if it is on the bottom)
JST-2-SMD-STANDARD = smd 1.6 x 3.4: NC1 -3.4,1.5; NC2 3.4,1.5 | smd 1 x 4.6: NEG -1,-3.7; POS 1,-3.7
SJ = smd 1.168 x 1.6: 1 -0.762,0; 2 0.762,0
C0603-ROUND = smd 0.898 x 1.1: 1 -0.889,0; 2 0.889,0
CHIPLED_0603 = smd 0.8 x 0.8: A 0,-0.75; C 0,0.75
SOD523 = smd 0.7 x 0.5: A 0.7,0; C -0.6,0
SOD-323 = smd 0.63 x 0.83: A 1.15,0; C -1.15,0
1X05M = drill 1.016 octagon: 1 -5.08,0; 2 -2.54,0; 3 0,0; 4 2.54,0; 5 5.08,0
1X14M = drill 1.016 octagon: 1 -16.51,0; 2 -13.97,0; 3 -11.43,0; 4 -8.89,0; 5 -6.35,0; 6 -3.81,0; 7 -1.27,0; 8 1.27,0; 9 3.81,0; 10 6.35,0; 11 8.89,0; 12 11.43,0; 13 13.97,0; 14 16.51,0
SWPA4030S = smd 1.1 x 3.4: P$1 -1.5,0; P$2 1.5,0
CD32 = smd 3.6 x 1.7: 1 0,1.15; 2 0,-1.15
1X02M = drill 1.016 octagon: 1 -1.27,0; 2 1.27,0
SOT23 = smd 1 x 1.4: 1 -0.95,-1.1; 2 0.95,-1.1; 3 0,1.1
R0603-ROUND = smd 0.898 x 1.1: 1 -0.889,0; 2 0.889,0
TACTILE-SWITCH-1101NE = smd 2.3 x 1.6: 1 -3.15,0; 2 3.15,0
MICROSD-PUSHPULL = smd 1.4 x 0.7: 1 10.57,-3.52; 2 10.57,-2.42; 3 10.57,-1.32; 4 10.57,-0.22; 5 10.57,0.88; 6 10.57,1.98; 7 10.57,3.08; 8 10.57,4.18; CD 10.57,5.28 | smd 1.4 x 1.2: GND1 9.9,6.53 | smd 1.2 x 1.4: GND2 9.9,-8.17 | smd 2.2 x 1.2: GND3 0.3,6.53; GND4 0.3,-9.07 | hole 1: -0.1,3.63; -0.1,-4.37
SOT23-5 = smd 0.55 x 1.2: 1 -0.95,-1.3; 2 0,-1.3; 3 0.95,-1.3; 4 0.95,1.3; 5 -0.95,1.3
SOT23-6L = smd 0.55 x 1.2: 1 -0.95,-1.3; 2 0,-1.3; 3 0.95,-1.3; 4 0.95,1.3; 5 0,1.3; 6 -0.95,1.3
SOT23-5' = smd 0.6 x 1.2: 1 -0.95,-1.306; 2 0,-1.306; 3 0.95,-1.306; 4 0.95,1.306; 5 -0.95,1.306
TQFP64-10X10 = smd 1.2 x 0.3: 1 -5.7,3.75; 2 -5.7,3.25; 3 -5.7,2.75; 4 -5.7,2.25; 5 -5.7,1.75; 6 -5.7,1.25; 7 -5.7,0.75; 8 -5.7,0.25; 9 -5.7,-0.25; 10 -5.7,-0.75; 11 -5.7,-1.25; 12 -5.7,-1.75; 13 -5.7,-2.25; 14 -5.7,-2.75; 15 -5.7,-3.25; 16 -5.7,-3.75; 33 5.7,-3.75; 34 5.7,-3.25; 35 5.7,-2.75; 36 5.7,-2.25; 37 5.7,-1.75; 38 5.7,-1.25; 39 5.7,-0.75; 40 5.7,-0.25; 41 5.7,0.25; 42 5.7,0.75; 43 5.7,1.25; 44 5.7,1.75; 45 5.7,2.25; 46 5.7,2.75; 47 5.7,3.25; 48 5.7,3.75 | smd 0.3 x 1.2: 17 -3.75,-5.7; 18 -3.25,-5.7; 19 -2.75,-5.7; 20 -2.25,-5.7; 21 -1.75,-5.7; 22 -1.25,-5.7; 23 -0.75,-5.7; 24 -0.25,-5.7; 25 0.25,-5.7; 26 0.75,-5.7; 27 1.25,-5.7; 28 1.75,-5.7; 29 2.25,-5.7; 30 2.75,-5.7; 31 3.25,-5.7; 32 3.75,-5.7; 49 3.75,5.7; 50 3.25,5.7; 51 2.75,5.7; 52 2.25,5.7; 53 1.75,5.7; 54 1.25,5.7; 55 0.75,5.7; 56 0.25,5.7; 57 -0.25,5.7; 58 -0.75,5.7; 59 -1.25,5.7; 60 -1.75,5.7; 61 -2.25,5.7; 62 -2.75,5.7; 63 -3.25,5.7; 64 -3.75,5.7
SOT23-3 = smd 0.8 x 0.9: 1 -0.95,-1; 2 0.95,-1; 3 0,1.1
USB-B-MICRO-SMD_V03 = smd 1.45 x 0.4: D+1 2.725,0; D-1 2.725,0.65; GND1 2.725,-1.3; ID1 2.725,-0.65; VBUS1 2.725,1.3 | smd 1.5 x 1.8: SHIELD1 0,3.685; SHIELD2 0,-3.685 | smd 1.5 x 2.5: SHIELD3 0,0 | hole 0.85: 2.2,1.9; 2.2,-1.9
ESP12SMD-NARROW = smd 3 x 1.5: ADC -6.988,1.25; CH_PD -6.988,-0.75; GND 6.988,-10.75; GPIO0 6.988,-4.75; GPIO2 6.988,-6.75; GPIO4 6.988,-2.75; GPIO5 6.988,-0.75; GPIO12 -6.988,-6.75; GPIO13 -6.988,-8.75; GPIO14 -6.988,-4.75; GPIO15 6.988,-8.75; GPIO16 -6.988,-2.75; RESET -6.988,3.25; RX 6.988,1.25; TX 6.988,3.25; VCC -6.988,-10.75
FC145 = smd 1.1 x 1.8: P$1 -1.6,0; P$2 1.6,0
IQG2520 = smd 0.925 x 0.825: P$1 -0.8,-0.6; P$2 0.8,-0.6; P$3 0.8,0.6; P$4 -0.8,0.6

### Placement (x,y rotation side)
BAT1  3.19,8.05 90 top
BCK  1.92,16.56 90 bottom
C1  11.32,6.66 0 top
C2  20.85,7.67 90 bottom
C3  20.46,8.44 90 top
C4  8.4,12.75 0 top
C5  11.19,19.1 0 top
C6  4.72,20.88 180 top
C7  19.19,16.82 90 top
C8  9.03,19.87 90 top
C9  35.83,11.99 270 top
C10  34.43,10.72 270 top
C11  34.31,14.02 90 top
C12  33.04,9.96 270 top
C13  30.75,9.07 180 top
C14  30.75,10.47 180 top
C15  32.91,14.02 270 top
C16  22.37,20.12 0 bottom
C17  38.63,17.2 0 bottom
C18  21.48,17.45 90 bottom
C19  22.24,11.36 90 bottom
C20  23.77,13.9 0 bottom
C34  10.18,7.04 0 bottom
C35  9.42,11.48 0 bottom
CHG  9.54,11.1 90 top
D1  19.19,5.64 90 top
D2  18.69,10.09 180 top
D3  11.57,12.75 180 top
D4  18.69,8.31 180 top
D5  7.64,15.8 270 bottom
D6  6.11,14.02 180 bottom
D7  6.11,20.5 180 bottom
D8  6.49,18.85 0 bottom
D14  15.77,5.26 0 bottom
DZ1  17.16,20.75 0 bottom
DZ2  25.54,17.45 0 bottom
ICSP  14.5,2.34 0 top
JP2  38.63,22.66 0 bottom
JP4  38.63,2.34 180 bottom
L1  4.72,14.91 0 top
L2  15.77,18.34 90 top
L3  9.16,15.8 270 top
LDEN  25.16,18.85 90 top
ON  10.69,22.66 180 top
PWR  22.62,17.96 90 top
Q1  15.77,8.05 0 top
Q2  12.97,9.71 270 bottom
Q3  16.53,10.59 0 bottom
Q4  9.42,14.15 270 bottom
Q5  12.84,16.06 180 bottom
Q6  4.97,16.69 270 bottom
Q7  19.83,12.25 180 bottom
Q8  16.78,17.07 270 bottom
R1  12.08,11.1 0 top
R2  14.37,10.21 90 top
R3  16.02,6.66 180 bottom
R4  19.07,7.67 90 bottom
R5  16.4,8.05 0 bottom
R6  14.37,13.39 180 bottom
R7  21.1,5.64 90 top
R8  18.05,5.64 270 top
R9  26.81,19.61 90 top
R10  12.84,18.47 0 bottom
R11  17.8,13.9 90 top
R12  11.19,20.75 0 top
R13  19.19,13.9 270 top
R14  7.64,19.87 90 top
R15  22.75,15.55 180 top
R16  22.75,11.86 0 top
R18  9.16,19.48 0 bottom
R19  26.81,19.48 90 bottom
R20  44.59,12.25 180 bottom
R21  41.67,16.44 90 bottom
R22  43.07,16.44 90 bottom
R23  44.09,9.07 90 bottom
R24  40.91,5.39 90 bottom
R25  41.93,8.56 0 bottom
R26  45.36,9.07 90 bottom
R27  19.83,14.66 0 bottom
R28  17.04,19.23 0 bottom
R29  35.83,18.6 90 top
R30  35.83,15.8 270 top
R31  6.11,22.91 0 bottom
RESEN  23.26,7.8 180 top
RESET  26.43,12.63 270 top
RX/PRG  22.62,14.28 90 top
SD  57.55,12.5 0 bottom
TX  22.62,10.59 90 top
U1  11.96,8.94 270 top
U2  4.72,18.72 90 top
U3  LC3406  [SOT23-5']  15.51,14.15 180 top
U4  32.78,11.74 0 bottom
U6  9.03,9.2 270 bottom
U$2  [FISHINO_MEDIUM]  16.91,20.88 0 top
U$3  [FISHINO_MEDIUM]  45.74,3.86 0 bottom
U$4  [FISHINO_MEDIUM]  28.47,16.06 0 top
USB  2.05,8.18 180 bottom
WIFI  49.17,12.5 270 top
XT1  23.13,17.33 90 bottom
XT2  24.15,11.86 270 bottom

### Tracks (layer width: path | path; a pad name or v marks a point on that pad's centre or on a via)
0  (via drill 0.41)
  Top 0.152: v29.35,4.88 29.23,4.88 31.01,3.1 31.01,1.83 31.64,1.2 40.53,1.2 41.67,2.34 JP4.9
  Bottom 0.152: U4.31 29.53,5.19 29.23,4.88 v29.35,4.88
3
  Bottom 0.152: U4.61 35.03,18.05 35.83,18.85 44.98,18.85 46.5,20.37 49.04,20.37 50.56,18.85 50.56,2.85 JP4.12
4
  Bottom 0.152: U4.60 34.53,18.06 35.7,19.23 44.85,19.23 46.37,20.75 49.17,20.75 50.94,18.98 50.94,3.99 JP4.13
6
  Bottom 0.152: U4.55 32.03,18.1 32.28,18.34 32.78,18.34 33.04,18.6 33.04,18.85 33.67,19.48 34.94,19.48 35.45,19.99 44.59,19.99 46.12,21.52 53.87,21.52 55.01,22.66 JP2.1
7  (via drill 0.41)
  Top 0.152: v32.15,18.98 33.16,18.98 33.55,19.36 33.93,19.36 34.43,19.87 34.43,20.75 34.82,21.14 35.96,21.14 36.21,21.39 51.2,21.39 52.47,22.66 JP2.2
  Bottom 0.152: U4.54 31.53,18.11 32.15,18.72 v32.15,18.98
9/SCK  (via drill 0.41)
  Top 0.152: v32.15,20.88 33.55,22.15 33.55,23.17 34.18,23.8 46.37,23.8 JP2.4
  Bottom 0.152: 27.2,20.63 R19.2 27.32,20.75 30.37,20.75 30.75,21.14 31.89,21.14 v32.15,20.88
!OFF  (via drill 0.41)
  Top 0.203: U2.4 3.39,19.67 v2.68,20.25
  Bottom 0.203: DZ1.C 18.31,22.65 17.16,23.8 6.11,23.8 R31.2 2.68,20.37 v2.68,20.25 | U4.45 25.96,13.99 25.16,14.79 22.12,14.79 20.46,16.18 20.46,18.21 19.58,19.1 R28.1
  Bottom 0.406: R28.1 17.92,20.37 DZ1.C
  Bottom 0.61: R28.1 17.92,17.81 Q8.1
+3V3  (via drill 0.41, 0.61)
  Top 0.406: v19.32,18.47 18.69,18.47 18.56,18.34
  Top 0.508: v31.64,15.04 31.64,16.82 32.53,17.71 34.05,17.71 R29.2 | R9.2 28.85,20.5 29.48,19.99 29.48,15.17 v29.61,15.04
  Top 0.61: C13.2 v28.97,9.07 27.96,9.07 27.96,12.88 29.61,14.53 v29.61,15.04 | WIFI.VCC 38.42,17.41 39.51,16.31 v40.28,16.31 40.28,13.77 42.69,11.36 v42.94,11.36 43.83,12.25 v48.15,12.25
  Top 0.813: R11.2 17.8,18.34 | 17.8,18.34 L2.2 | 17.8,18.34 18.56,18.34 C7.2 | WIFI.VCC R29.2
  Top 1.016: 17.8,18.34 17.8,20.63 23.64,20.63 24.02,21.01 27.07,21.01 | 27.07,21.01 R9.2 | 27.07,21.01 27.07,22.53 JP2.12
  Bottom 0.152: R23.2 42.94,11.1 v42.94,11.36
  Bottom 0.254: U4.35 28.8,8.99 v28.97,9.07
  Bottom 0.305: v48.15,12.25 48.12,12.28 SD.4 45.52,12.28 R20.2
  Bottom 0.356: v19.32,18.47 19.83,17.96 Q7.3
  Bottom 0.61: R22.2 R21.2 40.28,17.33 | 40.28,17.33 39.64,17.33 C17.1 | v40.28,16.31 40.28,17.33 | v31.64,15.04 v29.61,15.04
  pour Top (no thermals): 19.96,16.82 19.96,21.14 16.02,21.14 16.02,16.44 18.31,16.44 18.31,16.82
+3V3CORE  (via drill 0.41)
  Top 0.61: C14.2 v28.97,10.47 | v32.4,8.05 33.04,8.69 C12.2 33.29,8.82 v34.31,8.82 34.43,8.94 C10.2 35.2,9.83 v35.7,10.34 35.83,10.47 C9.2 | ICSP.2 13.35,3.74 15.51,3.74 16.53,4.75 17.04,4.75 | 17.04,4.75 R8.2 19.19,4.75 | 19.19,4.75 20.08,4.75 | 20.08,4.75 R7.1 | D1.C 19.19,4.75 | 17.04,4.75 v17.04,5.26 | v20.08,5.26 20.08,4.75
  Top 0.813: C11.2 34.31,15.8 v34.05,16.06
  Bottom 0.254: 28.97,10.49 v28.97,10.47 | U4.57 33.03,16.57 33.55,16.06 v34.05,16.06 | U4.26 32.03,7.69 v32.4,8.05 | U4.19 35.53,7.59 v34.31,8.82 | U4.10 36.35,10.99 v35.7,10.34
  Bottom 0.305: v28.97,10.47 28.95,10.49 U4.38 26.07,10.49 25.29,9.71
  Bottom 0.356: 21.02,13.85 21.02,14.23 R27.1
  Bottom 0.406: 22.12,7.8 22.12,6.53 20.85,5.26 D14.C v17.04,5.26 | 25.29,9.71 24.02,9.71 22.12,7.8 | 21.02,13.85 Q7.2 20.78,10.15 22.12,8.82 22.12,7.8
  Bottom 0.61: 28.97,10.49 29.97,10.49 v32.4,8.05 | v34.05,16.06 34.05,11.99 v35.7,10.34
  pour Bottom (no thermals): 28.47,6.91 37.23,6.91 37.61,7.29 37.61,16.18 37.23,16.56 28.34,16.56 27.96,16.18 27.96,7.42
+5V  (via drill 0.41)
  Top 0.305: 12.72,11.1 11.96,10.34 11.96,9.71 13.26,8.41 U1.4
  Top 0.406: R1.2 12.72,11.1 | U3.1 16.46,14.22 v16.53,14.28
  Top 0.61: U3.4 14.14,12.75 D3.C 12.08,12.75 C5.2 | 12.97,12.51 13.09,12.51 v13.61,11.86
  Top 0.813: D3.C 12.97,12.51 R1.2 | C5.2 R12.2 12.59,20.75 13.73,21.9 13.73,22.66 14.62,23.55 21.23,23.55 JP2.14
  Bottom 0.406: 16.53,11.86 v16.53,14.28 | v13.61,11.86 15.26,11.86 | 15.26,11.86 16.53,11.86 | 16.53,11.86 Q3.3 | R6.2 15.26,11.86
  pour Top (no thermals): 11.57,11.99 13.35,11.99 13.35,21.39 11.57,21.39
  pour Top (no thermals): 23.26,21.9 21.23,21.9 21.23,22.66 15.13,22.66 15.13,20.5 11.57,20.5 11.57,21.39 12.59,21.39 13.23,22.02 13.23,23.93 23.26,23.93
  pour Top (no thermals): 11.57,13.52 14.88,13.52 14.88,12.12 11.57,12.12
A1
  Bottom 0.152: U4.28 31.03,4.65 29.86,3.48 28.34,3.48 JP4.3
A2
  Bottom 0.152: U4.27 31.53,4.14 JP4.4
A3
  Bottom 0.152: U4.24 33.03,3.1 JP4.5
A4
  Bottom 0.152: U4.23 33.53,3.62 JP4.6
A5
  Bottom 0.152: U4.22 34.03,4.26 34.82,3.48 35.45,3.48 36.59,2.34 JP4.7
A6
  Bottom 0.152: U4.21 34.53,4.27 34.94,3.86 35.7,3.86 36.09,3.48 38.75,3.48 JP4.8
AREF
  Bottom 0.152: U4.16 38.48,4.39 39.39,3.48 40.53,3.48 41.17,2.85 41.17,1.7 40.66,1.2 23,1.2 22.12,2.09 JP4.1
BATOFF  (via drill 0.41)
  Top 0.203: v13.61,7.04 13.84,7.04 Q1.1
  Bottom 0.203: D5.C 7.73,16.31 8.65,16.31 9.42,15.55 9.42,14.4 9.67,14.15 11.19,14.15 12.46,12.88 12.46,11.23 12.97,10.72 12.97,7.67 v13.61,7.04
  Bottom 0.406: R18.2 7.73,19.48 D8.C 7.09,18.66 Q6.1
  Bottom 0.61: Q6.1 6.4,17.64 D5.C
D+
  Bottom 0.152: U4.37 26.33,9.99 25.54,9.2 24.4,9.2 22.75,7.55 22.75,4.75 22.24,4.24 7.51,4.24 6.37,5.39 6.37,7.29 5.48,8.18 USB.D+1
D-
  Bottom 0.152: U4.36 26.34,9.49 25.67,8.82 24.53,8.82 23.13,7.42 23.13,4.63 22.37,3.86 7.38,3.86 5.99,5.26 5.99,7.04 5.49,7.53 USB.D-1
ESPBMODE  (via drill 0.41)
  Top 0.152: WIFI.GPIO0 44.47,5.56 v44.47,7.42 43.32,8.56 38.88,8.56 37.74,7.42 v36.21,7.42
  Bottom 0.152: v44.47,7.42 44.09,7.8 R23.1 44.09,8.56 | U4.18 36.03,7.37 v36.21,7.42
ESPCHPD  (via drill 0.41)
  Top 0.356: WIFI.CH_PD 48.42,17.34 47.9,16.82 v45.48,16.82
  Bottom 0.152: v45.48,16.82 45.1,16.82 44.72,16.44 41.93,16.44 41.67,16.18 R21.1 40.86,14.99 U4.2
ESPGPIO2/XPGC  (via drill 0.41)
  Top 0.152: WIFI.GPIO2 42.42,7.4 v42.44,7.42
  Bottom 0.152: R25.1 42.82,7.8 v42.44,7.42
ESPGPIO4/XPGD  (via drill 0.41)
  Top 0.152: WIFI.GPIO4 46.37,5.56 v46.37,7.55
  Bottom 0.152: R26.1 45.99,7.55 v46.37,7.55
ESPGPIO5/REMOTERESET  (via drill 0.41)
  Top 0.152: WIFI.GPIO5 48.42,3.75 48.15,3.48 31.77,3.48 29.74,5.51 27.83,5.51 27.58,5.26 v27.58,4.88 | v24.91,7.67 23.64,7.67 RESEN.1 RESEN.2 21.86,8.44 19.41,8.44 D4.C
  Bottom 0.152: v27.58,4.88 24.91,7.55 v24.91,7.67
ESPRDY  (via drill 0.41)
  Top 0.356: v44.59,17.33 44.85,17.58 45.86,17.58 46.42,18.13 WIFI.GPIO16
  Bottom 0.152: v44.59,17.33 43.83,18.09 38.88,18.09 38.63,17.83 38.63,15.63 U4.1
ESPRESET  (via drill 0.41)
  Top 0.356: WIFI.RESET 52.42,17.78 50.44,15.8 v45.48,15.8
  Bottom 0.152: U4.3 42.52,14.49 43.07,15.04 R22.1 43.32,15.8 v45.48,15.8
ESPSS  (via drill 0.41)
  Top 0.152: WIFI.GPIO15 40.66,5.75 40.66,6.78 v41.29,7.42
  Bottom 0.152: R24.2 40.91,7.04 v41.29,7.42 41.8,7.93 41.8,10.34 41.55,10.59 39.77,10.59 39.16,9.99 U4.12
FB
  Top 0.406: U2.3 6.43,19.67 7.38,20.63 R14.2 C8.2 R12.1
FB2
  Top 0.406: R13.2 R11.1 16.46,13.01 U3.5
GND  (via drill 0.41, 0.61, 0.81)
  Top 0.406: R13.1 C7.1 | 17.04,11.1 17.04,7.27 Q1.2 | C6.1 5.1,20.88 4.97,20.75 4.97,18.98 5.22,18.72 U2.2 7.38,18.72 R14.1 | 26.05,15.04 26.43,15.42 RESET.1 25.14,17.07 20.72,17.07
  Top 0.508: JP2.11 29.74,21.52 30.24,21.01 30.24,17.45 30.62,17.07 30.62,14.15 31.64,13.13
  Top 0.61: 20.72,15.93 20.72,17.07 20.72,17.96 | C7.1 20.72,15.93 | U1.2 11.45,8.94 11.96,8.44 v11.96,7.55 11.96,7.04 C1.2 | WIFI.GND 38.42,7.08 39.13,7.8 v39.9,7.8 | 20.72,10.98 20.59,11.1 17.04,11.1 16.53,11.1 15.51,12.12 v15.51,14.53 U3.2 | BAT1.NEG 8.64,7.05 8.64,6.8 10.05,5.39 11.83,5.39 12.21,5.77 C1.2 | BAT1.NC2 BAT1.NC1 | C1.2 12.21,6.4 | 20.72,17.96 20.72,19.1 v20.85,19.23 | PWR.C 20.72,17.96 | 20.72,15.93 20.72,14.28 | 20.72,14.28 20.72,13.13 | 20.72,13.13 20.72,10.98 | TX.C 21.1,10.59 20.72,10.98 | RX/PRG.C 20.72,14.28 | R30.2 C9.1 | v22.24,13.13 20.72,13.13 | 31.64,8.82 31.39,8.56 31.39,7.67 32.02,7.04 33.29,7.04 v34.05,7.8
  Top 0.813: C14.1 C13.1 31.64,8.82 | C12.1 32.02,10.85 C14.1 | v36.98,10.22 37.11,10.34 v37.11,11.87 37.11,12.88 C9.1 35.58,13.13 C11.1 | v35.96,4.63 v37.1,4.63 37.53,4.63 WIFI.GND | BAT1.NC1 2.05,5.01 v2.05,6.4 3.07,7.42 6.65,7.42 BAT1.NEG | R14.1 C8.1 9.54,18.98 | 9.54,18.98 10.18,18.98 C5.1 10.3,18.6 v10.69,18.21 | 9.54,18.98 9.42,18.85 v9.42,18.21 9.42,17.56 L3.P$1 | C14.1 31.64,11.86 | 31.64,11.86 31.64,13.13 C15.2 C11.1 | v28.97,11.86 31.64,11.86 | C10.1 34.31,11.74 C11.1
  Bottom 0.305: U4.41 28.85,11.99 v28.97,11.86 | U4.25 32.53,6.92 33.42,7.8 v34.05,7.8 34.18,7.8 35.03,6.95 U4.20 35.03,4.92 35.32,4.63 v35.96,4.63 | U4.9 37.49,11.49 v37.11,11.87 | 36.97,10.09 v36.98,10.22
  Bottom 0.406: USB.GND1 2.27,9.48 2.11,9.64 | Q5.2 13.79,18.66 | v11.96,7.55 11.96,7.8 10.03,9.72 U6.1 10.3,10.42 C35.1 | C20.2 v22.24,13.13 C19.2 | 25.93,24.44 25.93,22.02 24.52,20.62 24.52,17.58 DZ2.A
  Bottom 0.61: 14.5,0.94 21.99,0.94 22.37,0.56 46.5,0.56 | 14.5,0.94 5.22,0.94 4.08,2.09 4.08,3.36 2.94,4.5 USB.SHIELD1 | 46.5,0.56 56.28,0.56 v57.17,1.45 57.25,1.53 SD.GND4 | ICSP.3 14.5,0.94 | 56.02,24.44 29.74,24.44 | C17.2 37.74,16.44 37.1,15.8 v37.1,11.87 v37.11,11.87 | 29.74,24.44 JP2.11 | 5.99,24.44 19.19,24.44 | 19.19,24.44 25.93,24.44 29.74,24.44 | C34.1 11.45,7.04 v11.96,7.55 | C16.2 21.48,19.23 | R10.1 13.79,18.66 13.73,18.66 13.73,19.61 | 10.05,18.21 R18.1 13.73,19.61 | 13.73,19.61 16.02,19.61 | 16.02,19.61 16.15,19.61 R28.2 | DZ1.A 16.02,20.75 16.02,19.61 | C2.2 R4.2 19.07,9.96 17.67,11.36 17.67,15.74 | 17.67,15.74 Q8.2 | 17.67,15.74 17.6,15.55 15.51,15.55 | Q5.2 13.79,16.76 15,15.55 15.51,15.55 | C18.2 21.48,19.23 | 21.48,19.23 v20.85,19.23 19.19,20.88 19.19,24.44 | 15.51,15.55 v15.51,14.53 | SD.6 49.11,14.48 49.29,14.66 | v46.25,1.07 46.25,0.82 46.5,0.56
  Bottom 0.813: 2.05,9.71 USB.SHIELD3 v2.05,6.41 v2.05,6.4 USB.SHIELD1 | USB.SHIELD2 v2.05,9.83 2.05,9.71 | 40.91,4.33 39.94,4.33 39.26,5.01 39.26,7.04 39.9,7.67 v39.9,7.8 | 40.91,4.33 SD.GND2 | R24.1 40.91,4.33 | v48.53,7.8 49.17,7.8 49.29,7.67 | SD.GND3 57.17,19.11 v57.17,21.9 57.17,23.29 56.02,24.44 | 2.05,9.71 2.11,9.64
  Bottom 1.016: SD.GND2 48.49,4.33 49.29,5.13 49.29,7.67 49.29,14.66 49.29,18.34 48.66,18.98 47.7,18.98 SD.GND1 | v8.15,18.21 10.05,18.21 v10.69,18.21 | 57.17,19.11 52.86,19.11 52.6,18.85 v52.6,15.8 v52.6,12.5 v52.6,9.2 52.6,5.26 53.36,4.5 54.25,4.5 54.75,3.99 56.69,3.99 SD.GND4
  pour Top (no thermals): 4.72,18.47 7.13,18.47 7.13,16.18 11.19,16.18 11.19,19.74 7,19.74 7,19.1 5.22,19.1 5.22,20.25 6.24,20.25 6.24,21.52 4.72,21.52
  pour Bottom (rank 3, no thermals): 0.02,0.05 0.02,25.07 61.74,25.07 61.74,0.05
  pour Top (rank 3, no thermals): 0.02,0.05 0.02,25.07 62.12,25.07 62.12,0.05
LONGRESET  (via drill 0.41)
  Top 0.152: R7.2 21.23,6.66 24.78,6.66 25.54,7.42 25.54,9.1 RESET.2 26.43,11.48 25.93,11.99 v25.93,12.12
  Top 0.406: C3.1 21.1,6.91 R7.2
  Bottom 0.203: U4.42 26.29,12.49 v25.93,12.12
MBAT  (via drill 0.41)
  Top 0.152: v24.15,6.02 21.86,6.02 21.48,5.64 20.59,5.64 19.96,6.28 v19.96,6.53
  Bottom 0.152: U4.30 30.03,4.67 29.61,4.24 25.29,4.24 24.15,5.39 v24.15,6.02 | C2.1 20.21,6.91 v19.96,6.53
  Bottom 0.406: R3.2 18.18,6.66 R4.1 C2.1
MCLR  (via drill 0.41)
  Top 0.152: ICSP.1 10.56,1.2 15.26,1.2 15.77,1.7 15.77,2.97 16.65,3.86 24.66,3.86 27.45,6.66 31.13,6.66 31.51,6.28 33.93,6.28 34.82,7.17 34.82,8.31 35.96,9.45 37.36,9.45 39.9,11.99 v39.9,12.63
  Top 0.254: ICSP.1 10.69,3.61 11.57,3.61 12.46,4.5 15.13,4.5 16.53,5.9 17.42,5.9 R8.1
  Top 0.406: R8.1 17.99,6.72 D4.A D2.A
  Bottom 0.152: U4.7 39.63,12.49 v39.9,12.63
N17690335
  Bottom 0.406: Q3.2 15.58,8.82 | 15.58,8.82 15.58,8.25 R5.2 | Q2.2 15.13,8.76 15.58,8.82
N$1  (via drill 0.41)
  Top 0.406: v13.23,6.15 14.11,5.26 v14.37,5.26
  Bottom 0.254: v13.23,6.15 10.18,6.15 C34.2 10.03,7.78 U6.2
  Bottom 0.406: D14.A v14.37,5.26
N$2  (via drill 0.41)
  Top 0.61: C15.1 33.16,15.42 v32.78,15.8
  Bottom 0.254: U4.56 32.53,16.06 v32.78,15.8
N$5
  Bottom 0.152: U4.47 25.6,14.99 25.16,15.42 23.56,15.42 XT1.P$1
  Bottom 0.406: XT1.P$1 22.32,15.73 C18.1
N$6
  Bottom 0.152: U4.48 25.73,15.49 25.04,16.18 24.53,16.18 23.13,17.58 XT1.P$2
  Bottom 0.406: C16.1 XT1.P$2
N$7
  Top 0.406: R2.2 15.77,9.71 Q1.3
N$10
  Top 0.406: R16.1 22.1,11.86 TX.A
N$13
  Top 0.152: LDEN.1 LDEN.2
  Top 0.406: R9.1 26.18,18.09 LDEN.1 25.42,17.96 PWR.A
N$14
  Top 0.406: R15.2 22.1,15.55 RX/PRG.A
N$20
  Top 0.406: R1.1 CHG.A
N$24
  Top 0.61: L3.P$2 9.29,14.17 C4.2 D3.A
  pour Top (no thermals): 8.65,12.12 11.19,12.12 11.19,15.42 7.13,15.42 7.13,13.64 8.65,13.64
N$34
  Bottom 0.356: Q8.3 18.81,17.07 19.07,16.82 19.07,14.91 R27.2 18.88,14.59 Q7.1
OSC1
  Bottom 0.152: U4.39 25.94,10.99 25.16,10.21 23.77,10.21 23.55,10.43 XT2.P$3
  Bottom 0.406: C19.1 23.55,10.47 XT2.P$3
OSC2
  Bottom 0.152: U4.40 25.54,11.49 24.62,12.41 XT2.P$1 | 24.62,13.86 C20.1
  Bottom 0.406: XT2.P$1 24.75,13.86 C20.1
PGC  (via drill 0.41)
  Top 0.152: ICSP.5 20.85,1.07 25.04,1.07 25.93,1.96 25.93,4.12 27.7,5.9 30.62,5.9 31.01,5.51 34.43,5.51 35.58,6.66 35.58,8.05 36.21,8.69 37.61,8.69 38.5,9.58 v40.15,9.58
  Bottom 0.152: U4.14 39.56,8.99 v40.15,9.58 40.15,9.45 R25.2
PGD  (via drill 0.41)
  Top 0.152: ICSP.4 17.67,2.34 18.81,3.48 24.78,3.48 27.58,6.28 30.88,6.28 31.26,5.9 34.18,5.9 35.2,6.91 35.2,8.18 36.09,9.07 37.48,9.07 39.13,10.72 41.17,10.72 | v43.96,10.98 43.45,10.98 43.2,10.72 41.17,10.72 | v41.17,9.83 41.17,10.72
  Bottom 0.152: U4.13 39.17,9.49 39.9,10.21 40.78,10.21 v41.17,9.83 | v43.96,10.98 44.34,10.98 R26.2
PROG
  Top 0.406: U1.5 13.07,9.96 13.7,9.32 R2.1
PWRGOOD  (via drill 0.41)
  Top 0.203: R30.1 35.83,16.44 v35.32,15.93
  Top 0.61: R29.1 R30.1
  Bottom 0.203: U4.62 35.53,16.14 v35.32,15.93
RESET  (via drill 0.41)
  Top 0.152: D1.A 19.19,6.91 18.69,7.42 18.69,9.49 D2.C | C3.2 20.72,9.32 21.1,8.94 23.89,8.94 24.53,9.58 24.53,11.61 25.67,12.75 26.94,12.75 28.47,14.28 28.47,16.56 28.97,17.07 28.97,19.36 v28.72,19.61 | v31.13,20.12 31.13,21.52 JP2.10
  Top 0.406: D2.C 19.7,9.45 19.83,9.32 C3.2
  Bottom 0.152: v28.72,19.61 30.37,19.61 30.88,20.12 v31.13,20.12
RXLED  (via drill 0.41)
  Top 0.152: R15.1 25.04,14.15 27.32,14.15 27.7,14.53 27.7,19.1 v27.83,19.23
  Bottom 0.152: U4.51 30.03,18.55 29.61,18.98 28.08,18.98 v27.83,19.23
SCK1
  Bottom 0.152: U4.50 29.53,18.16 29.1,18.6 R19.1
  Bottom 0.406: R19.1 26.81,17.57 DZ2.C
SCK2  (via drill 0.41)
  Top 0.356: WIFI.GPIO14 44.42,18.29 43.58,17.45 43.58,16.69 45.61,14.66 v45.61,14.28
  Bottom 0.152: SD.5 46.51,13.38 v45.61,14.28 45.48,14.15 39.51,14.15 39.35,13.99 U4.4
SCL1/12/SCL
  Bottom 0.152: U4.44 28.06,13.49 28.47,13.9 28.47,15.93 28.08,16.31 26.05,16.31 25.54,16.82 25.54,20.25 26.43,21.14 30.24,21.14 30.62,21.52 38.75,21.52 JP2.7
SDA1/11/SDA
  Bottom 0.152: U4.43 28.06,12.99 28.85,13.77 28.85,16.06 28.21,16.69 26.18,16.69 25.93,16.94 25.93,18.98 26.56,19.48 27.2,19.48 27.96,20.25 30.37,20.25 30.88,20.75 31.39,20.75 31.89,20.25 32.4,20.25 33.29,21.14 40.91,21.14 JP2.6
SDCS
  Bottom 0.152: U4.8 43.7,11.99 R20.1 45.1,10.85 45.74,10.85 46.51,10.08 SD.2
SDI1/10/MISO  (via drill 0.41)
  Top 0.152: v33.8,18.72 35.07,19.99 v35.07,20.5
  Bottom 0.152: U4.58 33.53,18.46 v33.8,18.72 | v35.07,20.5 35.32,20.75 43.07,20.75 JP2.5
SDI2/MISO2  (via drill 0.41)
  Top 0.356: WIFI.GPIO12 42.42,16.71 44.09,15.04 v44.09,14.79 44.09,14.4 v44.98,13.52
  Bottom 0.152: SD.7 46.28,15.58 45.74,15.04 44.34,15.04 v44.09,14.79 | U4.5 39.23,13.49 39.39,13.64 44.85,13.64 v44.98,13.52
SDO1/8/MOSI
  Bottom 0.152: U4.46 27.91,14.49 28.08,14.66 28.08,15.8 27.96,15.93 25.93,15.93 25.16,16.69 25.16,20.37 26.31,21.52 30.12,21.52 31.01,22.41 31.01,23.29 31.51,23.8 48.91,23.8 JP2.3
SDO2/MOSI2  (via drill 0.41)
  Top 0.356: v42.69,12.75 42.69,15.29 40.42,17.57 WIFI.GPIO13
  Bottom 0.152: SD.3 45.28,11.18 44.59,11.86 44.59,12.75 44.09,13.26 42.69,13.26 | U4.6 39.24,12.99 39.51,13.26 42.69,13.26 | v42.69,12.75 42.69,13.26
STAT2
  Top 0.305: U1.1 10.24,9.89 9.03,11.1 CHG.C
SW
  Top 0.61: C4.1 6.49,12.75 6.24,13.01 6.24,14.89 L1.P$2 6.02,15.11 U2.1
  pour Top (no thermals): 4.72,18.09 6.75,18.09 6.75,13.26 8.27,13.26 8.27,12.12 4.72,12.12
SW2
  Top 0.61: U3.3 14.56,18.29 L2.1
  pour Top (no thermals): 14.88,14.53 14.88,16.56 15.51,16.56 15.51,20.25 13.73,20.25 13.73,14.53
TXLED  (via drill 0.41)
  Top 0.152: v28.34,17.71 28.08,17.45 28.08,14.4 26.81,13.13 25.16,13.13 23.89,11.86 R16.2
  Bottom 0.152: U4.49 28.61,17.44 v28.34,17.71
U3RX/ESPTX  (via drill 0.41)
  Top 0.152: WIFI.TX 52.42,7.09 49.17,10.34 42.31,10.34 41.8,9.83 41.8,9.32 41.42,8.94 38.37,8.94 37.48,8.05 v36.97,8.05
  Bottom 0.152: U4.15 37.41,8.49 v36.97,8.05
U3TX/ESPRX  (via drill 0.41)
  Top 0.152: v42.82,9.71 47.9,9.71 50.42,7.19 WIFI.RX
  Bottom 0.152: U4.11 39.15,10.49 39.64,10.98 42.05,10.98 42.82,10.21 v42.82,9.71
U4RX/13/RX  (via drill 0.41)
  Top 0.152: v31.26,18.72 31.26,19.23 31.77,19.74 33.67,19.74 34.05,20.12 34.05,20.88 34.69,21.52 35.7,21.52 36.85,22.66 JP2.8
  Bottom 0.152: U4.53 31.03,18.5 v31.26,18.72
USBID  (via drill 0.41)
  Top 0.152: v26.18,7.8 26.18,7.17 24.15,5.13 22.37,5.13 v22.12,5.39
  Bottom 0.152: 15.77,4.63 7.64,4.63 6.75,5.51 6.75,7.55 5.46,8.83 USB.ID1 | 15.77,4.63 21.35,4.63 v22.12,5.39 | U4.33 26.37,7.99 v26.18,7.8 | R5.1 16.78,8.05 16.02,7.29 16.02,6.15 15.77,5.9 15.77,4.63
  Bottom 0.203: Q5.1 11.89,16.62 12.46,16.06 13.48,16.06 14.37,15.17 14.37,13.01 13.86,12.5 13.23,12.5 12.97,12.25 12.97,11.48 13.8,10.66 Q2.1 17.1,10.66 17.48,10.28 Q3.1
  Bottom 0.406: Q5.1 11.89,18.66 R10.2 | Q3.1 17.54,8.8 R5.1
USBSW
  Bottom 0.305: 13.08,14.85 Q5.3
  Bottom 0.406: Q5.3 13.48,14.45 R6.1
  Bottom 0.61: Q5.3 12.83,15.1 Q4.1
VIN  (via drill 0.61)
  Top 0.61: v16.02,21.9 v20.34,21.9
  Bottom 0.305: D8.A 5.79,19.79 D7.A
  Bottom 0.406: D7.A 7.39,20.63
  Bottom 0.61: 7.39,20.63 13.86,20.63 15.13,21.9 v16.02,21.9 | v20.34,21.9 20.85,21.39 23.51,21.39 24.66,22.53 JP2.13
VLIPO  (via drill 0.41, 0.61)
  Top 0.406: v5.86,10.47 5.86,10.09 BAT1.POS | v4.97,11.36 v7.76,11.36
  Top 0.61: BAT1.POS 8.27,9.05 | 8.27,9.05 8.8,9.05 9.86,7.99 U1.3 10.43,7.77 C1.1 | v8.27,8.18 8.27,9.05
  Bottom 0.152: BCK.1 BCK.2
  Bottom 0.254: R3.1 15.26,6.53 14.62,6.53 13.48,5.39 9.67,5.39 8.27,6.78 v8.27,8.18
  Bottom 0.406: v5.86,10.47 5.86,11.61 3.87,13.6 Q6.3 BCK.2 | U6.3 8.53,9.79 C35.2 | C35.2 8.4,11.36 | v7.76,11.36 7.89,11.48 C35.2 | v4.97,11.36 1.92,14.4 BCK.1
VOR
  Bottom 0.356: D7.C 4.96,15.8 | 4.96,15.8 D6.C | Q6.2 6.01,15.8 4.96,15.8
  Bottom 0.406: D7.C 4.96,21.51 5.22,21.77 8.02,21.77 8.4,21.39 10.69,21.39 ON.1
VSEPIC
  Top 0.61: 3.83,21.14 1.54,21.14 1.54,18.6 | 1.54,18.6 1.54,15.55 2.18,14.91 L1.P$1 | U2.5 1.67,18.72 1.54,18.6
  Top 0.813: ON.2 4.34,22.66 3.83,22.15 3.83,21.14 C6.2
  Bottom 0.406: R31.1 9.16,22.91 ON.2
  pour Top (no thermals): 1.03,12.88 4.34,12.88 4.34,21.9 10.43,21.9 10.43,23.93 2.2,23.93 arc90 1.03,22.76
VUSB  (via drill 0.81)
  Top 1.27: v8.02,5.64 6.37,3.61 6.37,2.34 | v5.61,2.34 6.37,2.34 | 6.37,2.34 v6.88,2.34
  Bottom 0.152: v6.88,2.34 8.02,3.48 22.5,3.48 23.51,4.5 23.51,7.29 24.71,8.49 U4.34 | USB.VBUS1 5.22,6.88
  Bottom 0.406: 5.22,6.88 5.22,5.77
  Bottom 0.61: v8.02,5.64 7.38,6.28 7.38,7.8 6.88,8.31 6.88,12.5 7.32,12.95 10.26,12.95 Q4.2 11.13,13.2 11.83,12.5 11.83,9.75 Q2.3
  Bottom 0.813: v5.61,2.34 5.22,2.72 5.22,5.77
  Bottom 1.27: v6.88,2.34 v5.61,2.34
VUSBSW
  Bottom 0.61: Q4.3 8.19,14.02 7.76,14.02 | 7.76,14.02 D6.A | D5.A 7.64,14.15 7.76,14.02
~1  (via drill 0.41)
  Top 0.152: v28.47,4.88 28.47,1.83 29.48,0.82 43.45,0.82 JP4.10
  Bottom 0.152: U4.32 28.99,6.04 28.47,5.51 v28.47,4.88
~2
  Bottom 0.152: U4.63 36.03,18.16 36.34,18.47 45.1,18.47 46.63,19.99 48.91,19.99 50.18,18.72 50.18,4.24 48.28,2.34 JP4.11
~5
  Bottom 0.152: U4.59 34.03,18.07 35.58,19.61 44.72,19.61 46.25,21.14 49.29,21.14 51.33,19.1 51.33,4.5 52.21,3.61 53.87,3.61 JP4.14
~DAC/A0
  Bottom 0.152: U4.29 30.53,4.66 29.74,3.86 26.18,3.86 JP4.2
~U4TX/14/TX  (via drill 0.41)
  Top 0.152: v33.42,20.37 33.42,21.26 JP2.9
  Bottom 0.152: U4.52 30.53,19.14 30.88,19.48 31.39,19.48 31.64,19.74 32.78,19.74 v33.42,20.37

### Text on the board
tNames: +5V | VIN | 3.3V | GND | RES | D14 | D13 | D12 | D11 | D10 | D9 | D8 | D7 | D6 | + | - | FISHINO PIRANHA | MCLR | 3V3C | GND | PGD | PGC | AREF | A0 | A1 | A2 | A3 | A4 | A5 | A6 | D0 | D1 | D2 | D3 | D4 | D5
bNames: Designed by Massimo Del Fedele | FISHINO | PIRANHA | WWW.FISHINO.COM | PIRANHA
